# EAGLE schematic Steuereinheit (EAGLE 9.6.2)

## Sheet 1 of 5: PINS
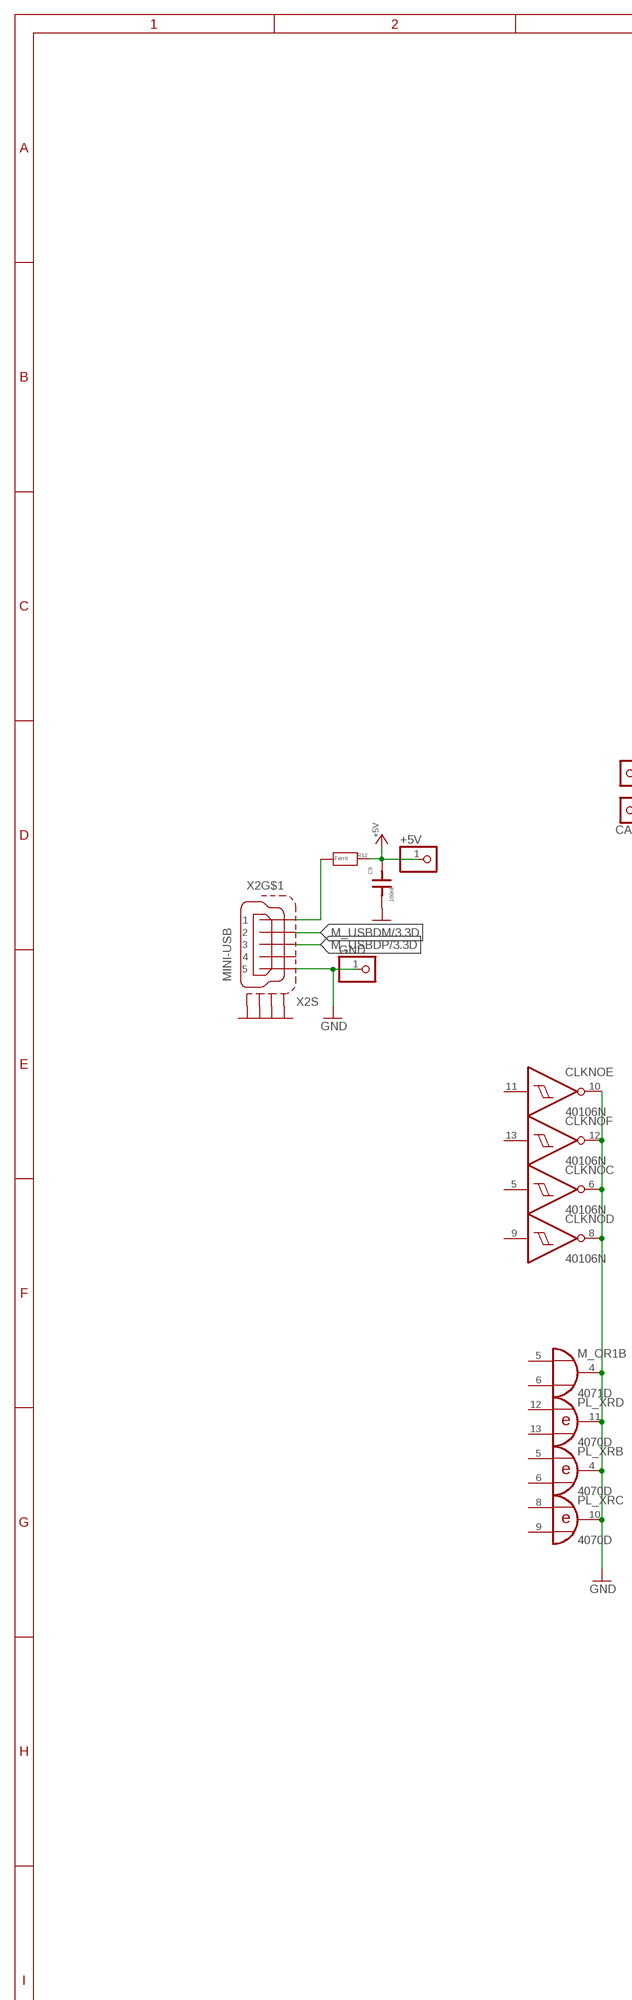
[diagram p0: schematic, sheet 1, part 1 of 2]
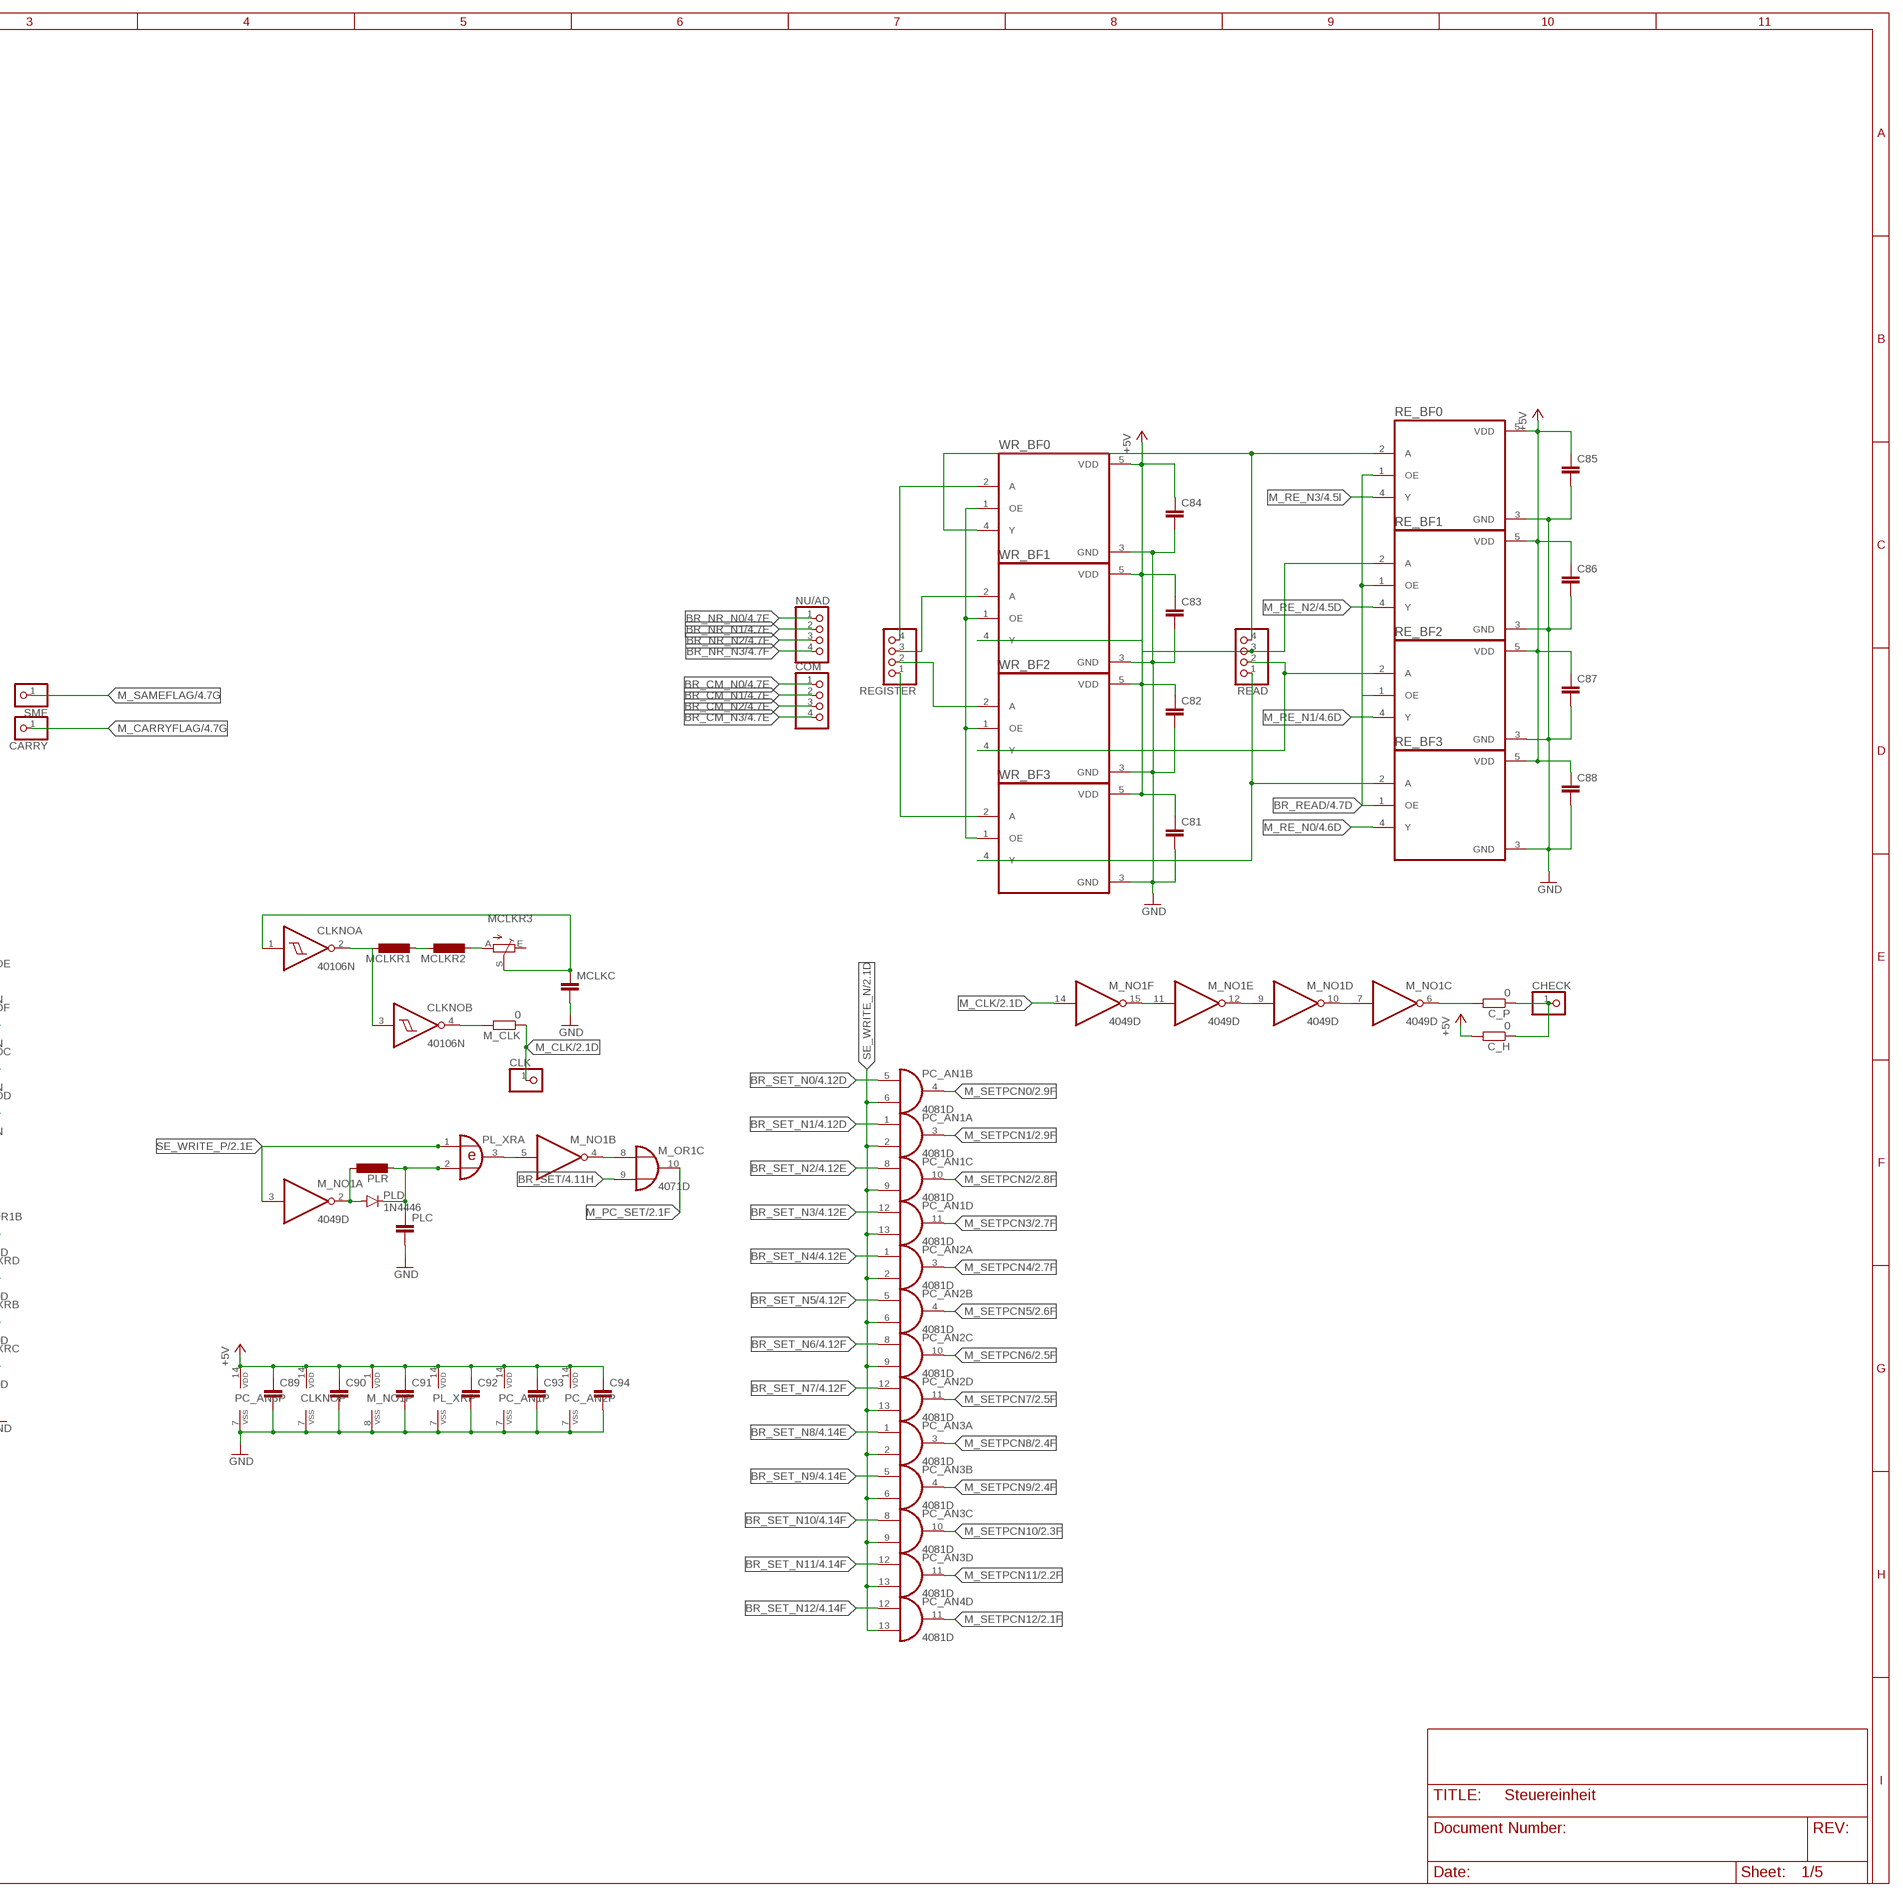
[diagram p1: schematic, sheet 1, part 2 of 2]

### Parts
+5V  PINHD-1X1  [1X01]
C9  100nF  C1  [0805F]
C81  C-EUC0805  [C0805]
C82  C-EUC0805  [C0805]
C83  C-EUC0805  [C0805]
C84  C-EUC0805  [C0805]
C85  C-EUC0805  [C0805]
C86  C-EUC0805  [C0805]
C87  C-EUC0805  [C0805]
C88  C-EUC0805  [C0805]
C89  C-EUC0805  [C0805]
C90  C-EUC0805  [C0805]
C91  C-EUC0805  [C0805]
C92  C-EUC0805  [C0805]
C93  C-EUC0805  [C0805]
C94  C-EUC0805  [C0805]
C_H  0  R-EU_R0805  [R0805]
C_P  0  R-EU_R0805  [R0805]
CARRY  PINHD-1X1  [1X01]
CHECK  PINHD-1X1  [1X01]
CLK  PINHD-1X1  [1X01]
CLKNO  40106N  [DIL14]
COM  PINHD-1X4  [1X04]
GND  PINHD-1X1  [1X01]
M_CLK  0  R-EU_R0805  [R0805]
M_NO1  4049D  [SO16]
M_OR1  4071D  [SO14]
MCLKC  C-EU025-030X050  [C025-030X050]
MCLKR1  L-EU0207/10  [0207/10]
MCLKR2  L-EU0207/10  [0207/10]
MCLKR3  TRIM_EU-CT6  [CT6]
NU/AD  PINHD-1X4  [1X04]
PC_AN1  4081D  [SO14]
PC_AN2  4081D  [SO14]
PC_AN3  4081D  [SO14]
PC_AN4  4081D  [SO14]
PL_XR  4070D  [SO14]
PLC  C-EU050-025X075  [C050-025X075]
PLD  1N4446  [DO35-10]
PLR  L-EU0207/10  [0207/10]
R12  Ferrit  R2  [1206]
RE_BF0  SN74LVC1G126DBVR  [SOT95P280X145-5N]
RE_BF1  SN74LVC1G126DBVR  [SOT95P280X145-5N]
RE_BF2  SN74LVC1G126DBVR  [SOT95P280X145-5N]
RE_BF3  SN74LVC1G126DBVR  [SOT95P280X145-5N]
READ  PINHD-1X4  [1X04]
REGISTER  PINHD-1X4  [1X04]
SMF  PINHD-1X1  [1X01]
WR_BF0  SN74LVC1G126DBVR  [SOT95P280X145-5N]
WR_BF1  SN74LVC1G126DBVR  [SOT95P280X145-5N]
WR_BF2  SN74LVC1G126DBVR  [SOT95P280X145-5N]
WR_BF3  SN74LVC1G126DBVR  [SOT95P280X145-5N]
X2  MINI-USB  MINI-USB-SCHIELD-32005-201  [32005-201]

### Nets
+5V: +5V.1 C9.2 C81.1 C82.1 C83.1 C84.1 C85.1 C86.1 C87.1 C88.1 C89.1 C90.1 C91.1 C92.1 C93.1 C94.1 C_H.2 CLKNO.14(P:VDD) M_NO1.1(P:VDD) PC_AN1.14(P:VDD) PC_AN2.14(P:VDD) PC_AN3.14(P:VDD) PL_XR.14(P:VDD) R12.2 RE_BF0.5(VDD) RE_BF1.5(VDD) RE_BF2.5(VDD) RE_BF3.5(VDD) WR_BF0.5(VDD) WR_BF1.5(VDD) WR_BF2.5(VDD) WR_BF3.5(VDD) ; also sheet 2,3,4,5
BR_CM_N0: COM.1 ; also sheet 4
BR_CM_N1: COM.2 ; also sheet 4
BR_CM_N2: COM.3 ; also sheet 4
BR_CM_N3: COM.4 ; also sheet 4
BR_NR_N0: NU/AD.1 ; also sheet 4
BR_NR_N1: NU/AD.2 ; also sheet 4
BR_NR_N2: NU/AD.3 ; also sheet 4
BR_NR_N3: NU/AD.4 ; also sheet 4
BR_READ: RE_BF0.1(OE) RE_BF1.1(OE) RE_BF2.1(OE) RE_BF3.1(OE) ; also sheet 4
BR_SET: M_OR1.9(C:I1) ; also sheet 4
BR_SET_N0: PC_AN1.5(B:I0) ; also sheet 4
BR_SET_N1: PC_AN1.1(A:I0) ; also sheet 4
BR_SET_N2: PC_AN1.8(C:I0) ; also sheet 4
BR_SET_N3: PC_AN1.12(D:I0) ; also sheet 4
BR_SET_N4: PC_AN2.1(A:I0) ; also sheet 4
BR_SET_N5: PC_AN2.5(B:I0) ; also sheet 4
BR_SET_N6: PC_AN2.8(C:I0) ; also sheet 4
BR_SET_N7: PC_AN2.12(D:I0) ; also sheet 4
BR_SET_N8: PC_AN3.1(A:I0) ; also sheet 4
BR_SET_N9: PC_AN3.5(B:I0) ; also sheet 4
BR_SET_N10: PC_AN3.8(C:I0) ; also sheet 4
BR_SET_N11: PC_AN3.12(D:I0) ; also sheet 4
BR_SET_N12: PC_AN4.12(D:I0) ; also sheet 4
GND: C9.1 C81.2 C82.2 C83.2 C84.2 C85.2 C86.2 C87.2 C88.2 C89.2 C90.2 C91.2 C92.2 C93.2 C94.2 CLKNO.6(C:O) CLKNO.7(P:VSS) CLKNO.8(D:O) CLKNO.10(E:O) CLKNO.12(F:O) GND.1 M_NO1.8(P:VSS) M_OR1.4(B:O) MCLKC.2 PC_AN1.7(P:VSS) PC_AN2.7(P:VSS) PC_AN3.7(P:VSS) PL_XR.4(B:O) PL_XR.7(P:VSS) PL_XR.10(C:O) PL_XR.11(D:O) PLC.2 RE_BF0.3(GND) RE_BF1.3(GND) RE_BF2.3(GND) RE_BF3.3(GND) WR_BF0.3(GND) WR_BF1.3(GND) WR_BF2.3(GND) WR_BF3.3(GND) X2.5 X2.M1(S:S1) X2.M2(S:S2) X2.M3(S:S3) X2.M4(S:S4) ; also sheet 2,3,4,5
M_CARRYFLAG: CARRY.1 ; also sheet 4
M_CLK: CLK.1 M_CLK.1 M_NO1.14(F:I) ; also sheet 2,3,4
M_PC_SET: M_OR1.10(C:O) ; also sheet 2
M_RE_N0: RE_BF3.4(Y) ; also sheet 4
M_RE_N1: RE_BF2.4(Y) ; also sheet 4
M_RE_N2: RE_BF1.4(Y) ; also sheet 4
M_RE_N3: RE_BF0.4(Y) ; also sheet 4
M_SAMEFLAG: SMF.1 ; also sheet 4
M_SETPCN0: PC_AN1.4(B:O) ; also sheet 2
M_SETPCN1: PC_AN1.3(A:O) ; also sheet 2
M_SETPCN2: PC_AN1.10(C:O) ; also sheet 2
M_SETPCN3: PC_AN1.11(D:O) ; also sheet 2
M_SETPCN4: PC_AN2.3(A:O) ; also sheet 2
M_SETPCN5: PC_AN2.4(B:O) ; also sheet 2
M_SETPCN6: PC_AN2.10(C:O) ; also sheet 2
M_SETPCN7: PC_AN2.11(D:O) ; also sheet 2
M_SETPCN8: PC_AN3.3(A:O) ; also sheet 2
M_SETPCN9: PC_AN3.4(B:O) ; also sheet 2
M_SETPCN10: PC_AN3.10(C:O) ; also sheet 2
M_SETPCN11: PC_AN3.11(D:O) ; also sheet 2
M_SETPCN12: PC_AN4.11(D:O) ; also sheet 2
M_USBDM: X2.2 ; also sheet 3
M_USBDP: X2.3 ; also sheet 3
N$177: CLKNO.4(B:O) M_CLK.2
N$179: C_P.2 M_NO1.6(C:O)
N$180: CLKNO.2(A:O) CLKNO.3(B:I) MCLKR1.1
N$181: C_H.1 C_P.1 CHECK.1
N$182: MCLKR2.2 MCLKR3.A
N$183: M_NO1.2(A:O) PLD.A PLR.1
N$184: PL_XR.2(A:I1) PLC.1 PLD.C PLR.2
N$186: RE_BF0.2(A) READ.4 WR_BF0.4(Y)
N$187: M_NO1.5(B:I) PL_XR.3(A:O)
N$188: RE_BF1.2(A) READ.3 WR_BF1.4(Y)
N$190: RE_BF2.2(A) READ.2 WR_BF2.4(Y)
N$192: RE_BF3.2(A) READ.1 WR_BF3.4(Y)
N$193: REGISTER.4 WR_BF0.2(A)
N$194: REGISTER.3 WR_BF1.2(A)
N$195: REGISTER.2 WR_BF2.2(A)
N$196: REGISTER.1 WR_BF3.2(A)
N$197: WR_BF0.1(OE) WR_BF1.1(OE) WR_BF2.1(OE) WR_BF3.1(OE)
N$198: M_NO1.4(B:O) M_OR1.8(C:I0)
N$199: CLKNO.1(A:I) MCLKC.1 MCLKR3.S
N$208: M_NO1.11(E:I) M_NO1.15(F:O)
N$209: M_NO1.9(D:I) M_NO1.12(E:O)
N$210: M_NO1.7(C:I) M_NO1.10(D:O)
N$212: MCLKR1.2 MCLKR2.1
SE_WRITE_N: PC_AN1.2(A:I1) PC_AN1.6(B:I1) PC_AN1.9(C:I1) PC_AN1.13(D:I1) PC_AN2.2(A:I1) PC_AN2.6(B:I1) PC_AN2.9(C:I1) PC_AN2.13(D:I1) PC_AN3.2(A:I1) PC_AN3.6(B:I1) PC_AN3.9(C:I1) PC_AN3.13(D:I1) PC_AN4.13(D:I1) ; also sheet 2,3,5
SE_WRITE_P: M_NO1.3(A:I) PL_XR.1(A:I0) ; also sheet 2,3,5
USB_4: R12.1 X2.1
Unconnected: CLKNO.5(C:I) CLKNO.9(D:I) CLKNO.11(E:I) CLKNO.13(F:I) M_OR1.5(B:I0) M_OR1.6(B:I1) MCLKR3.E PL_XR.5(B:I0) PL_XR.6(B:I1) PL_XR.8(C:I0) PL_XR.9(C:I1) PL_XR.12(D:I0) PL_XR.13(D:I1) X2.4

## Sheet 2 of 5: ProgrammCounter
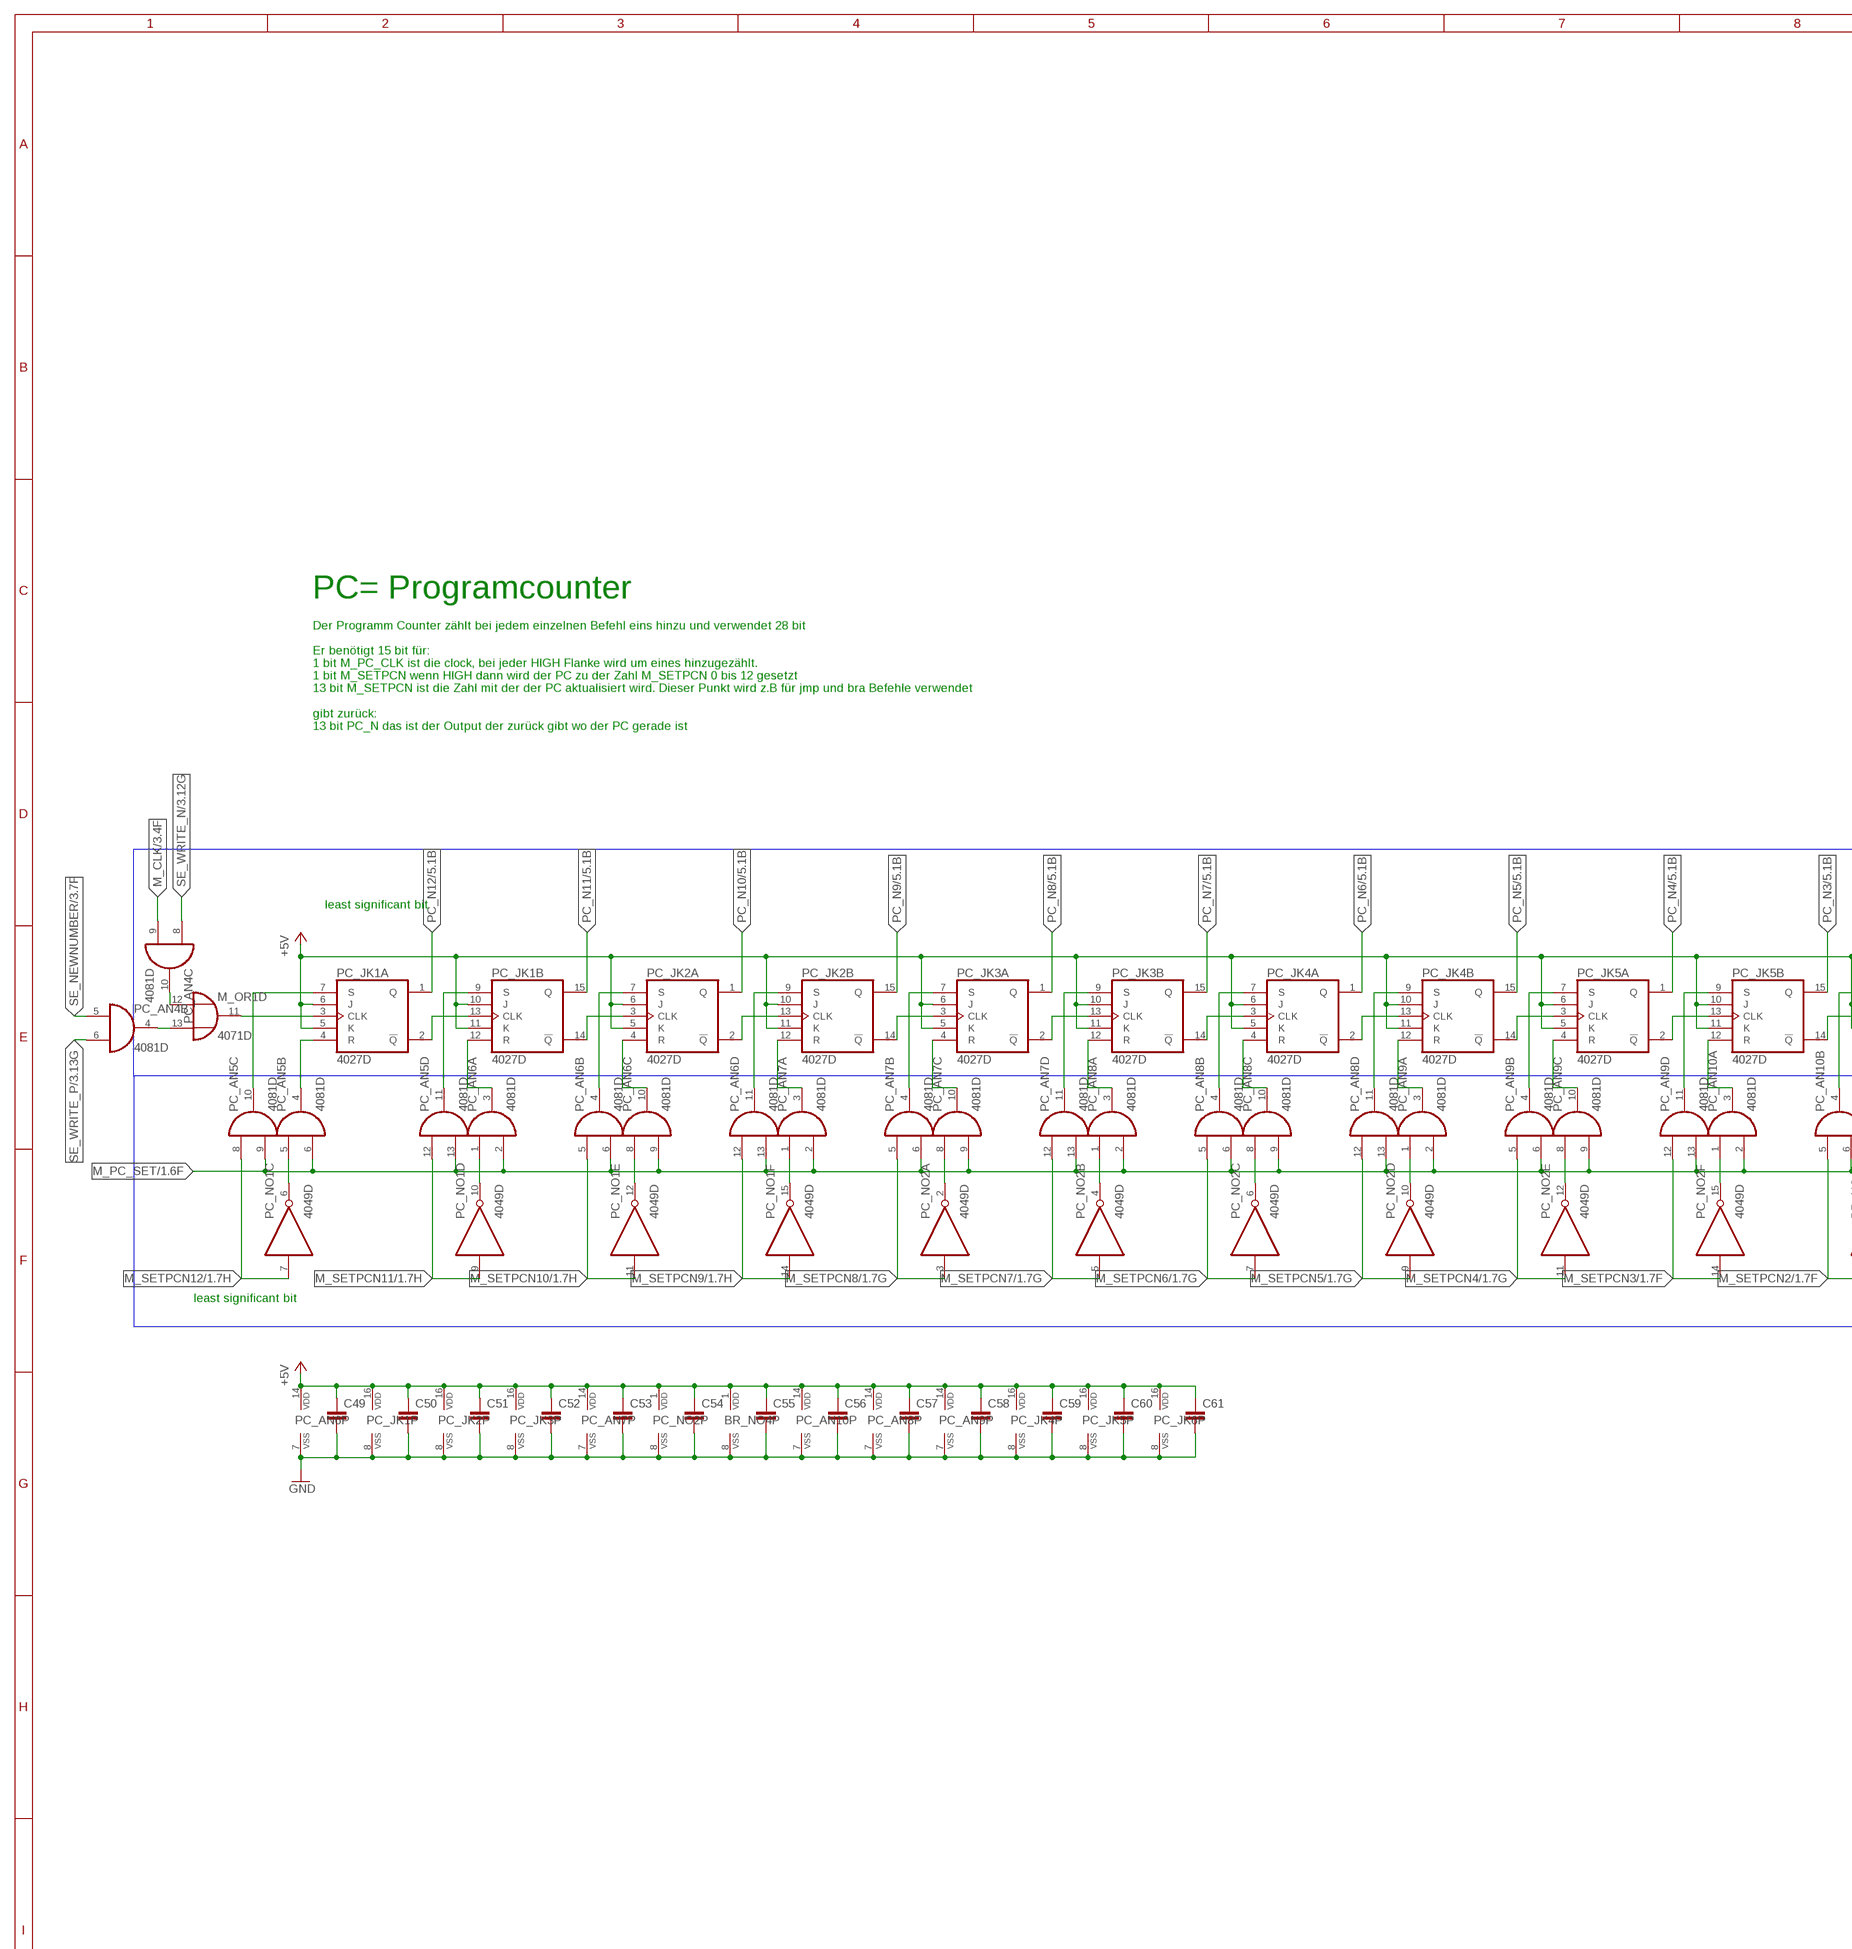
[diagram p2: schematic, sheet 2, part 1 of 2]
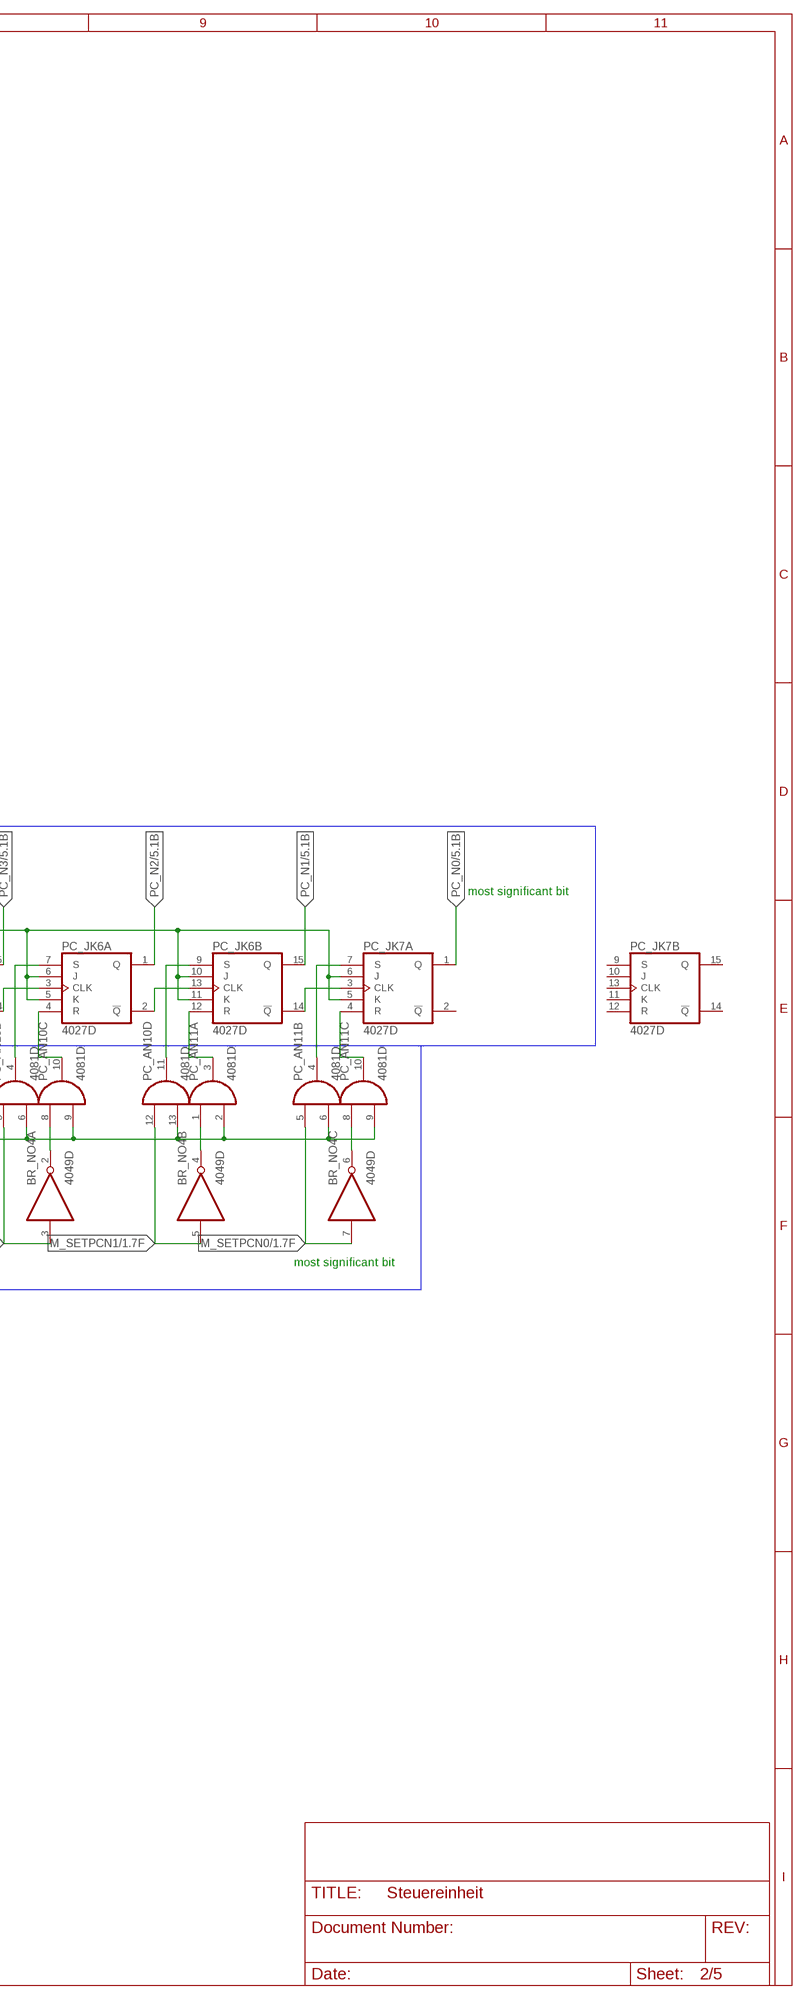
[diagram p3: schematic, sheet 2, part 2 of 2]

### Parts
BR_NO4  4049D  [SO16]
C49  C-EUC0805  [C0805]
C50  C-EUC0805  [C0805]
C51  C-EUC0805  [C0805]
C52  C-EUC0805  [C0805]
C53  C-EUC0805  [C0805]
C54  C-EUC0805  [C0805]
C55  C-EUC0805  [C0805]
C56  C-EUC0805  [C0805]
C57  C-EUC0805  [C0805]
C58  C-EUC0805  [C0805]
C59  C-EUC0805  [C0805]
C60  C-EUC0805  [C0805]
C61  C-EUC0805  [C0805]
PC_AN5  4081D  [SO14]
PC_AN6  4081D  [SO14]
PC_AN7  4081D  [SO14]
PC_AN8  4081D  [SO14]
PC_AN9  4081D  [SO14]
PC_AN10  4081D  [SO14]
PC_AN11  4081D  [SO14]
PC_JK1  4027D  [SO16]
PC_JK2  4027D  [SO16]
PC_JK3  4027D  [SO16]
PC_JK4  4027D  [SO16]
PC_JK5  4027D  [SO16]
PC_JK6  4027D  [SO16]
PC_JK7  4027D  [SO16]
PC_NO1  4049D  [SO16]
PC_NO2  4049D  [SO16]

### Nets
+5V: BR_NO4.1(P:VDD) C49.1 C50.1 C51.1 C52.1 C53.1 C54.1 C55.1 C56.1 C57.1 C58.1 C59.1 C60.1 C61.1 PC_AN6.14(P:VDD) PC_AN7.14(P:VDD) PC_AN8.14(P:VDD) PC_AN9.14(P:VDD) PC_AN10.14(P:VDD) PC_JK1.5(A:K) PC_JK1.6(A:J) PC_JK1.10(B:J) PC_JK1.11(B:K) PC_JK1.16(P:VDD) PC_JK2.5(A:K) PC_JK2.6(A:J) PC_JK2.10(B:J) PC_JK2.11(B:K) PC_JK2.16(P:VDD) PC_JK3.5(A:K) PC_JK3.6(A:J) PC_JK3.10(B:J) PC_JK3.11(B:K) PC_JK3.16(P:VDD) PC_JK4.5(A:K) PC_JK4.6(A:J) PC_JK4.10(B:J) PC_JK4.11(B:K) PC_JK4.16(P:VDD) PC_JK5.5(A:K) PC_JK5.6(A:J) PC_JK5.10(B:J) PC_JK5.11(B:K) PC_JK5.16(P:VDD) PC_JK6.5(A:K) PC_JK6.6(A:J) PC_JK6.10(B:J) PC_JK6.11(B:K) PC_JK6.16(P:VDD) PC_JK7.5(A:K) PC_JK7.6(A:J) PC_NO2.1(P:VDD) ; also sheet 1,3,4,5
GND: BR_NO4.8(P:VSS) C49.2 C50.2 C51.2 C52.2 C53.2 C54.2 C55.2 C56.2 C57.2 C58.2 C59.2 C60.2 C61.2 PC_AN6.7(P:VSS) PC_AN7.7(P:VSS) PC_AN8.7(P:VSS) PC_AN9.7(P:VSS) PC_AN10.7(P:VSS) PC_JK1.8(P:VSS) PC_JK2.8(P:VSS) PC_JK3.8(P:VSS) PC_JK4.8(P:VSS) PC_JK5.8(P:VSS) PC_JK6.8(P:VSS) PC_NO2.8(P:VSS) ; also sheet 1,3,4,5
M_CLK: PC_AN4.9(C:I1) ; also sheet 1,3,4
M_PC_SET: PC_AN5.6(B:I1) PC_AN5.9(C:I1) PC_AN5.13(D:I1) PC_AN6.2(A:I1) PC_AN6.6(B:I1) PC_AN6.9(C:I1) PC_AN6.13(D:I1) PC_AN7.2(A:I1) PC_AN7.6(B:I1) PC_AN7.9(C:I1) PC_AN7.13(D:I1) PC_AN8.2(A:I1) PC_AN8.6(B:I1) PC_AN8.9(C:I1) PC_AN8.13(D:I1) PC_AN9.2(A:I1) PC_AN9.6(B:I1) PC_AN9.9(C:I1) PC_AN9.13(D:I1) PC_AN10.2(A:I1) PC_AN10.6(B:I1) PC_AN10.9(C:I1) PC_AN10.13(D:I1) PC_AN11.2(A:I1) PC_AN11.6(B:I1) PC_AN11.9(C:I1) ; also sheet 1
M_SETPCN0: BR_NO4.7(C:I) PC_AN11.5(B:I0) ; also sheet 1
M_SETPCN1: BR_NO4.5(B:I) PC_AN10.12(D:I0) ; also sheet 1
M_SETPCN2: BR_NO4.3(A:I) PC_AN10.5(B:I0) ; also sheet 1
M_SETPCN3: PC_AN9.12(D:I0) PC_NO2.14(F:I) ; also sheet 1
M_SETPCN4: PC_AN9.5(B:I0) PC_NO2.11(E:I) ; also sheet 1
M_SETPCN5: PC_AN8.12(D:I0) PC_NO2.9(D:I) ; also sheet 1
M_SETPCN6: PC_AN8.5(B:I0) PC_NO2.7(C:I) ; also sheet 1
M_SETPCN7: PC_AN7.12(D:I0) PC_NO2.5(B:I) ; also sheet 1
M_SETPCN8: PC_AN7.5(B:I0) PC_NO2.3(A:I) ; also sheet 1
M_SETPCN9: PC_AN6.12(D:I0) PC_NO1.14(F:I) ; also sheet 1
M_SETPCN10: PC_AN6.5(B:I0) PC_NO1.11(E:I) ; also sheet 1
M_SETPCN11: PC_AN5.12(D:I0) PC_NO1.9(D:I) ; also sheet 1
M_SETPCN12: PC_AN5.8(C:I0) PC_NO1.7(C:I) ; also sheet 1
N$40: PC_JK1.2(A:!Q) PC_JK1.13(B:CLK)
N$50: PC_JK1.14(B:!Q) PC_JK2.3(A:CLK)
N$51: PC_JK2.2(A:!Q) PC_JK2.13(B:CLK)
N$52: PC_JK2.14(B:!Q) PC_JK3.3(A:CLK)
N$53: PC_JK3.2(A:!Q) PC_JK3.13(B:CLK)
N$54: PC_JK3.14(B:!Q) PC_JK4.3(A:CLK)
N$55: PC_JK4.2(A:!Q) PC_JK4.13(B:CLK)
N$56: PC_JK4.14(B:!Q) PC_JK5.3(A:CLK)
N$57: PC_JK5.2(A:!Q) PC_JK5.13(B:CLK)
N$58: PC_JK5.14(B:!Q) PC_JK6.3(A:CLK)
N$59: PC_JK6.2(A:!Q) PC_JK6.13(B:CLK)
N$60: PC_JK6.14(B:!Q) PC_JK7.3(A:CLK)
N$62: PC_AN5.10(C:O) PC_JK1.7(A:S)
N$63: PC_AN5.4(B:O) PC_JK1.4(A:R)
N$64: PC_AN5.11(D:O) PC_JK1.9(B:S)
N$65: PC_AN6.3(A:O) PC_JK1.12(B:R)
N$66: PC_AN6.4(B:O) PC_JK2.7(A:S)
N$67: PC_AN6.10(C:O) PC_JK2.4(A:R)
N$68: PC_AN6.11(D:O) PC_JK2.9(B:S)
N$69: PC_AN7.3(A:O) PC_JK2.12(B:R)
N$70: PC_AN7.4(B:O) PC_JK3.7(A:S)
N$71: PC_AN7.10(C:O) PC_JK3.4(A:R)
N$72: PC_AN7.11(D:O) PC_JK3.9(B:S)
N$73: PC_AN8.3(A:O) PC_JK3.12(B:R)
N$74: PC_AN8.4(B:O) PC_JK4.7(A:S)
N$75: PC_AN8.10(C:O) PC_JK4.4(A:R)
N$76: PC_AN8.11(D:O) PC_JK4.9(B:S)
N$77: PC_AN9.3(A:O) PC_JK4.12(B:R)
N$78: PC_AN9.4(B:O) PC_JK5.7(A:S)
N$79: PC_AN9.10(C:O) PC_JK5.4(A:R)
N$80: PC_AN9.11(D:O) PC_JK5.9(B:S)
N$81: PC_AN10.3(A:O) PC_JK5.12(B:R)
N$82: PC_AN10.4(B:O) PC_JK6.7(A:S)
N$83: PC_AN10.10(C:O) PC_JK6.4(A:R)
N$84: PC_AN10.11(D:O) PC_JK6.9(B:S)
N$85: PC_AN11.3(A:O) PC_JK6.12(B:R)
N$86: PC_AN11.4(B:O) PC_JK7.7(A:S)
N$87: PC_AN11.10(C:O) PC_JK7.4(A:R)
N$88: PC_AN5.5(B:I0) PC_NO1.6(C:O)
N$91: PC_AN6.1(A:I0) PC_NO1.10(D:O)
N$93: PC_AN6.8(C:I0) PC_NO1.12(E:O)
N$95: PC_AN7.1(A:I0) PC_NO1.15(F:O)
N$97: PC_AN7.8(C:I0) PC_NO2.2(A:O)
N$99: PC_AN8.1(A:I0) PC_NO2.4(B:O)
N$101: PC_AN8.8(C:I0) PC_NO2.6(C:O)
N$103: PC_AN9.1(A:I0) PC_NO2.10(D:O)
N$105: PC_AN9.8(C:I0) PC_NO2.12(E:O)
N$107: PC_AN10.1(A:I0) PC_NO2.15(F:O)
N$109: BR_NO4.2(A:O) PC_AN10.8(C:I0)
N$111: BR_NO4.4(B:O) PC_AN11.1(A:I0)
N$113: BR_NO4.6(C:O) PC_AN11.8(C:I0)
N$185: M_OR1.13(D:I1) PC_AN4.4(B:O)
N$189: M_OR1.11(D:O) PC_JK1.3(A:CLK)
N$191: M_OR1.12(D:I0) PC_AN4.10(C:O)
PC_N0: PC_JK7.1(A:Q) ; also sheet 5
PC_N1: PC_JK6.15(B:Q) ; also sheet 5
PC_N2: PC_JK6.1(A:Q) ; also sheet 5
PC_N3: PC_JK5.15(B:Q) ; also sheet 5
PC_N4: PC_JK5.1(A:Q) ; also sheet 5
PC_N5: PC_JK4.15(B:Q) ; also sheet 5
PC_N6: PC_JK4.1(A:Q) ; also sheet 5
PC_N7: PC_JK3.15(B:Q) ; also sheet 5
PC_N8: PC_JK3.1(A:Q) ; also sheet 5
PC_N9: PC_JK2.15(B:Q) ; also sheet 5
PC_N10: PC_JK2.1(A:Q) ; also sheet 5
PC_N11: PC_JK1.15(B:Q) ; also sheet 5
PC_N12: PC_JK1.1(A:Q) ; also sheet 5
SE_NEWNUMBER: PC_AN4.5(B:I0) ; also sheet 3
SE_WRITE_N: PC_AN4.8(C:I0) ; also sheet 1,3,5
SE_WRITE_P: PC_AN4.6(B:I1) ; also sheet 1,3,5
Unconnected: PC_JK7.2(A:!Q) PC_JK7.9(B:S) PC_JK7.10(B:J) PC_JK7.11(B:K) PC_JK7.12(B:R) PC_JK7.13(B:CLK) PC_JK7.14(B:!Q) PC_JK7.15(B:Q)

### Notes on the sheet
- PC= Programcounter
- Der Programm Counter zählt bei jedem einzelnen Befehl eins hinzu und verwendet 28 bit
  
  Er benötigt 15 bit für:
  1 bit M_PC_CLK ist die clock, bei jeder HIGH Flanke wird um eines hinzugezählt.
  1 bit M_SETPCN wenn HIGH dann wird der PC zu der Zahl M_SETPCN 0 bis 12 gesetzt
  13 bit M_SETPCN ist die Zahl mit der der PC aktualisiert wird. Dieser Punkt wird z.B für jmp und bra Befehle verwendet
  
  gibt zurück:
  13 bit PC_N das ist der Output der zurück gibt wo der PC gerade ist
- least significant bit
- most significant bit
- least significant bit | most significant bit

## Sheet 3 of 5: Serielle
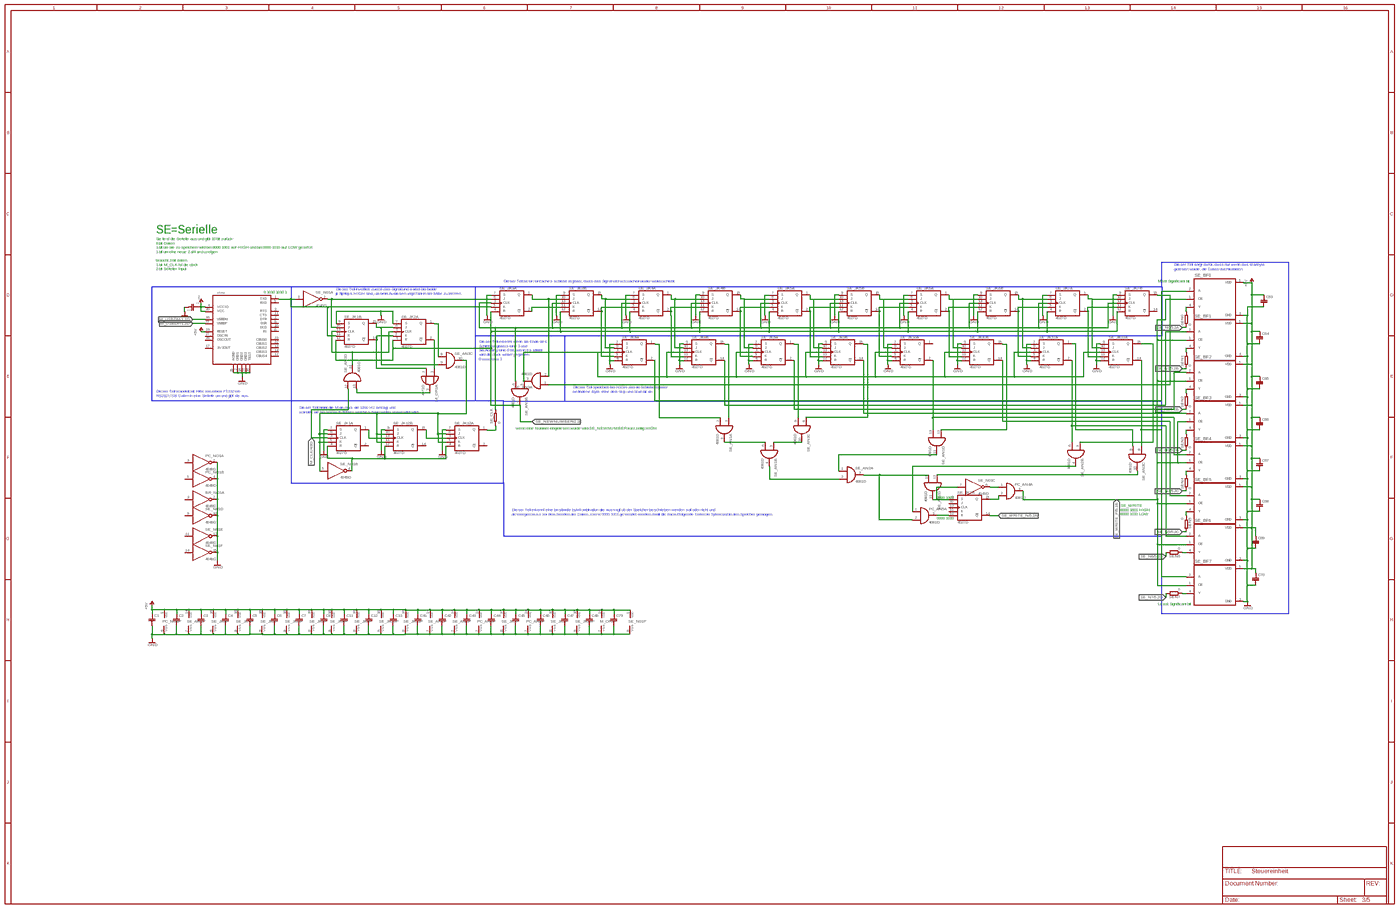
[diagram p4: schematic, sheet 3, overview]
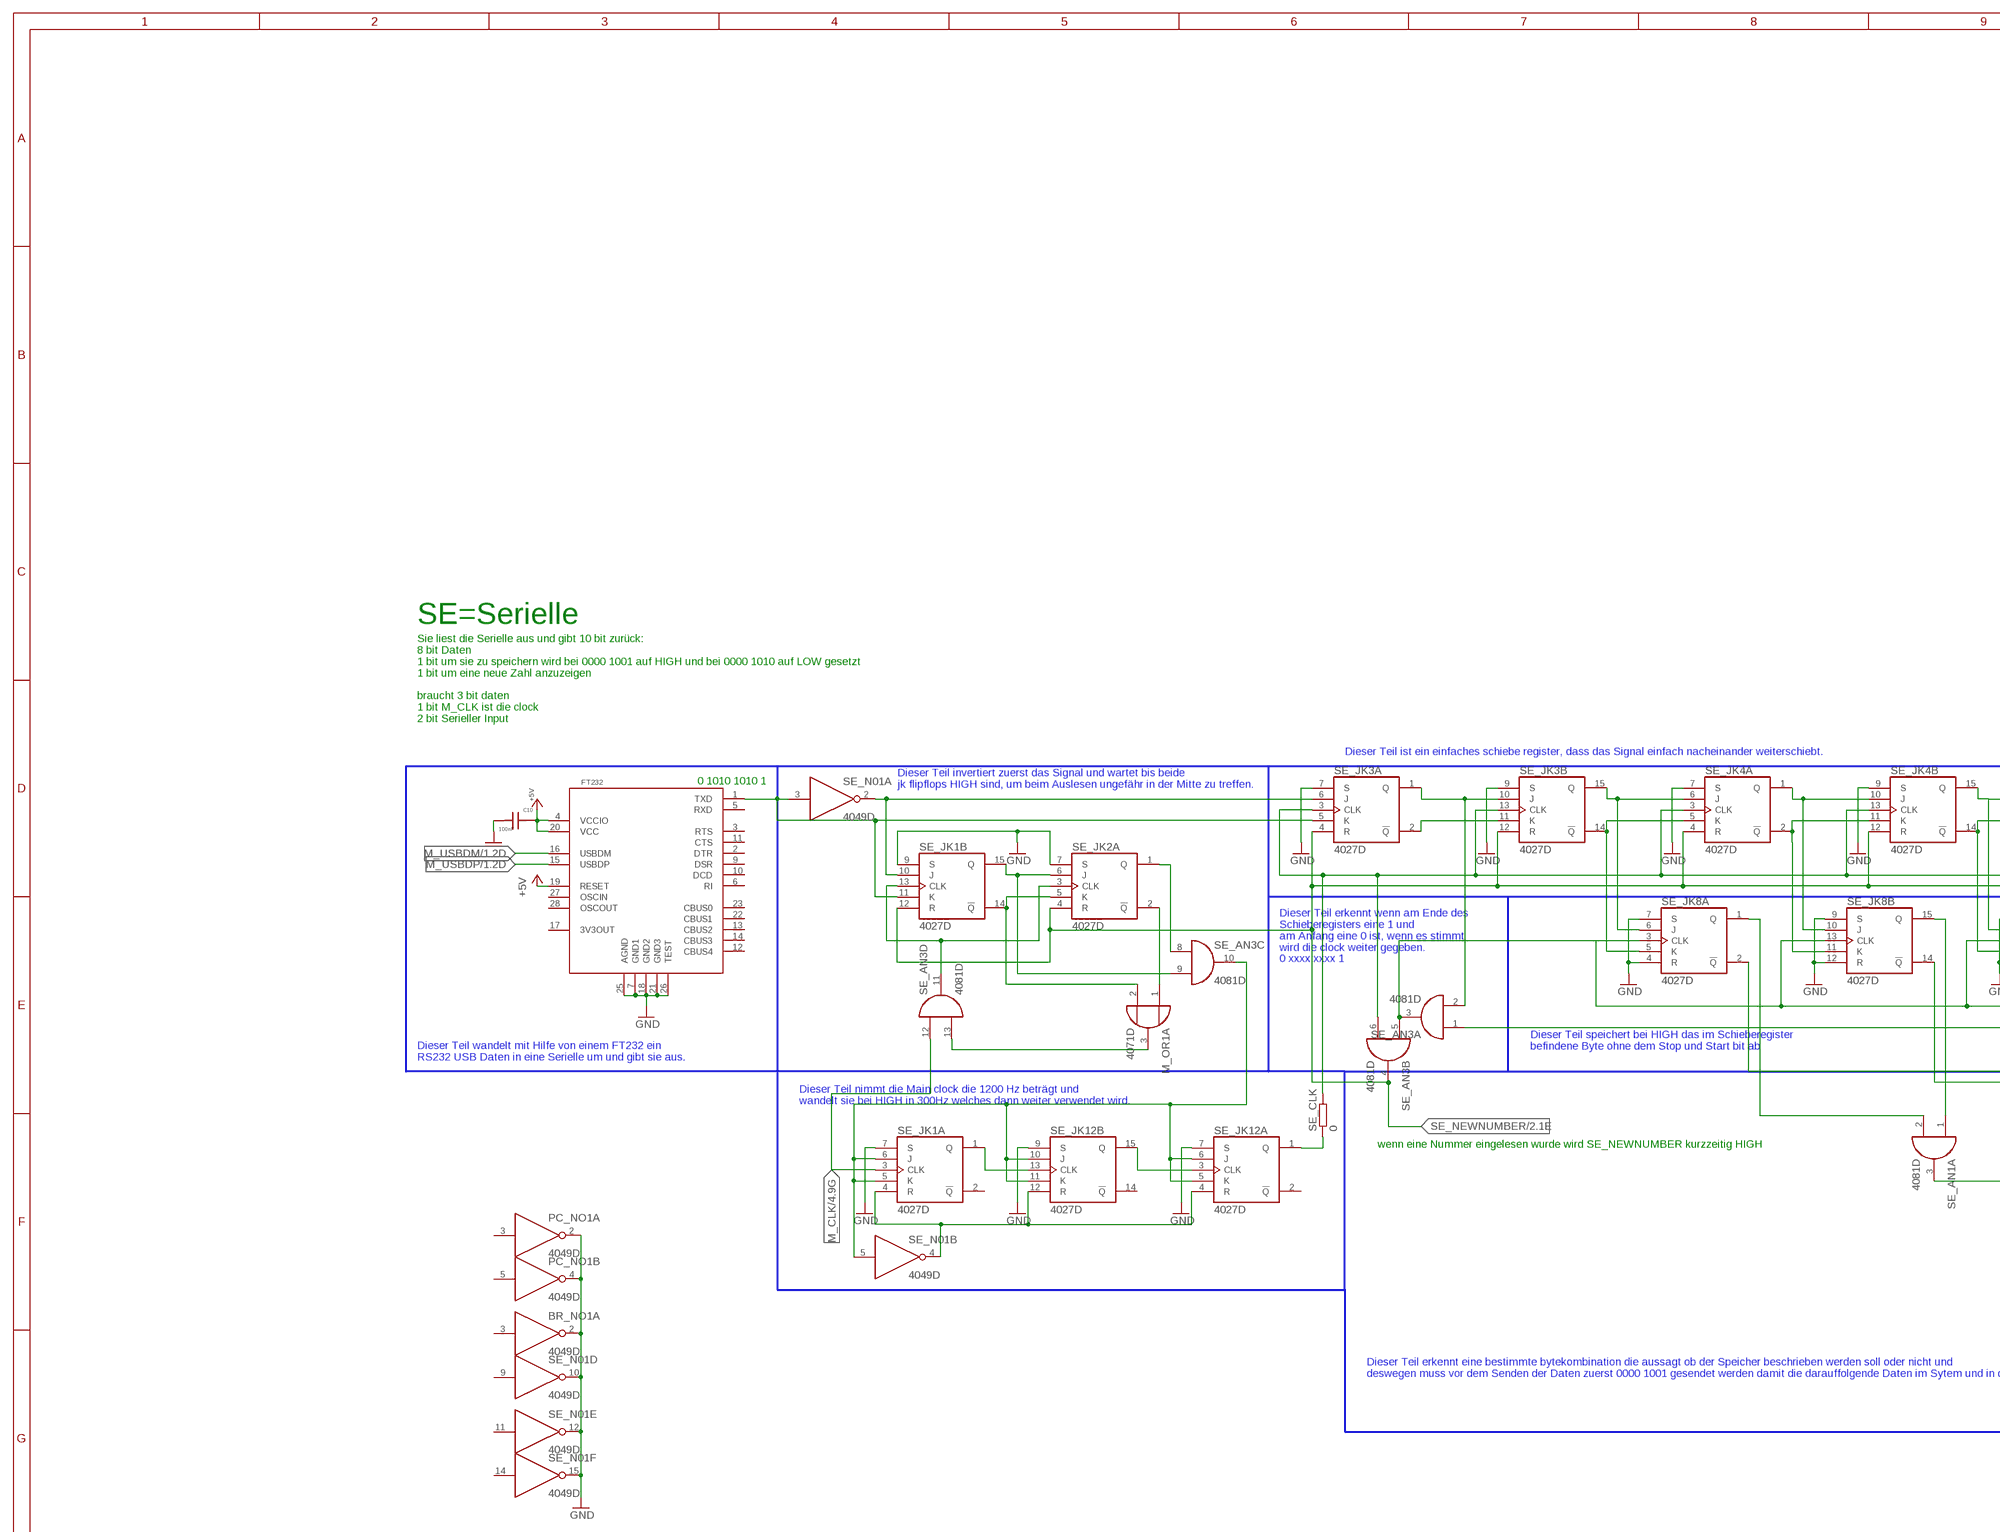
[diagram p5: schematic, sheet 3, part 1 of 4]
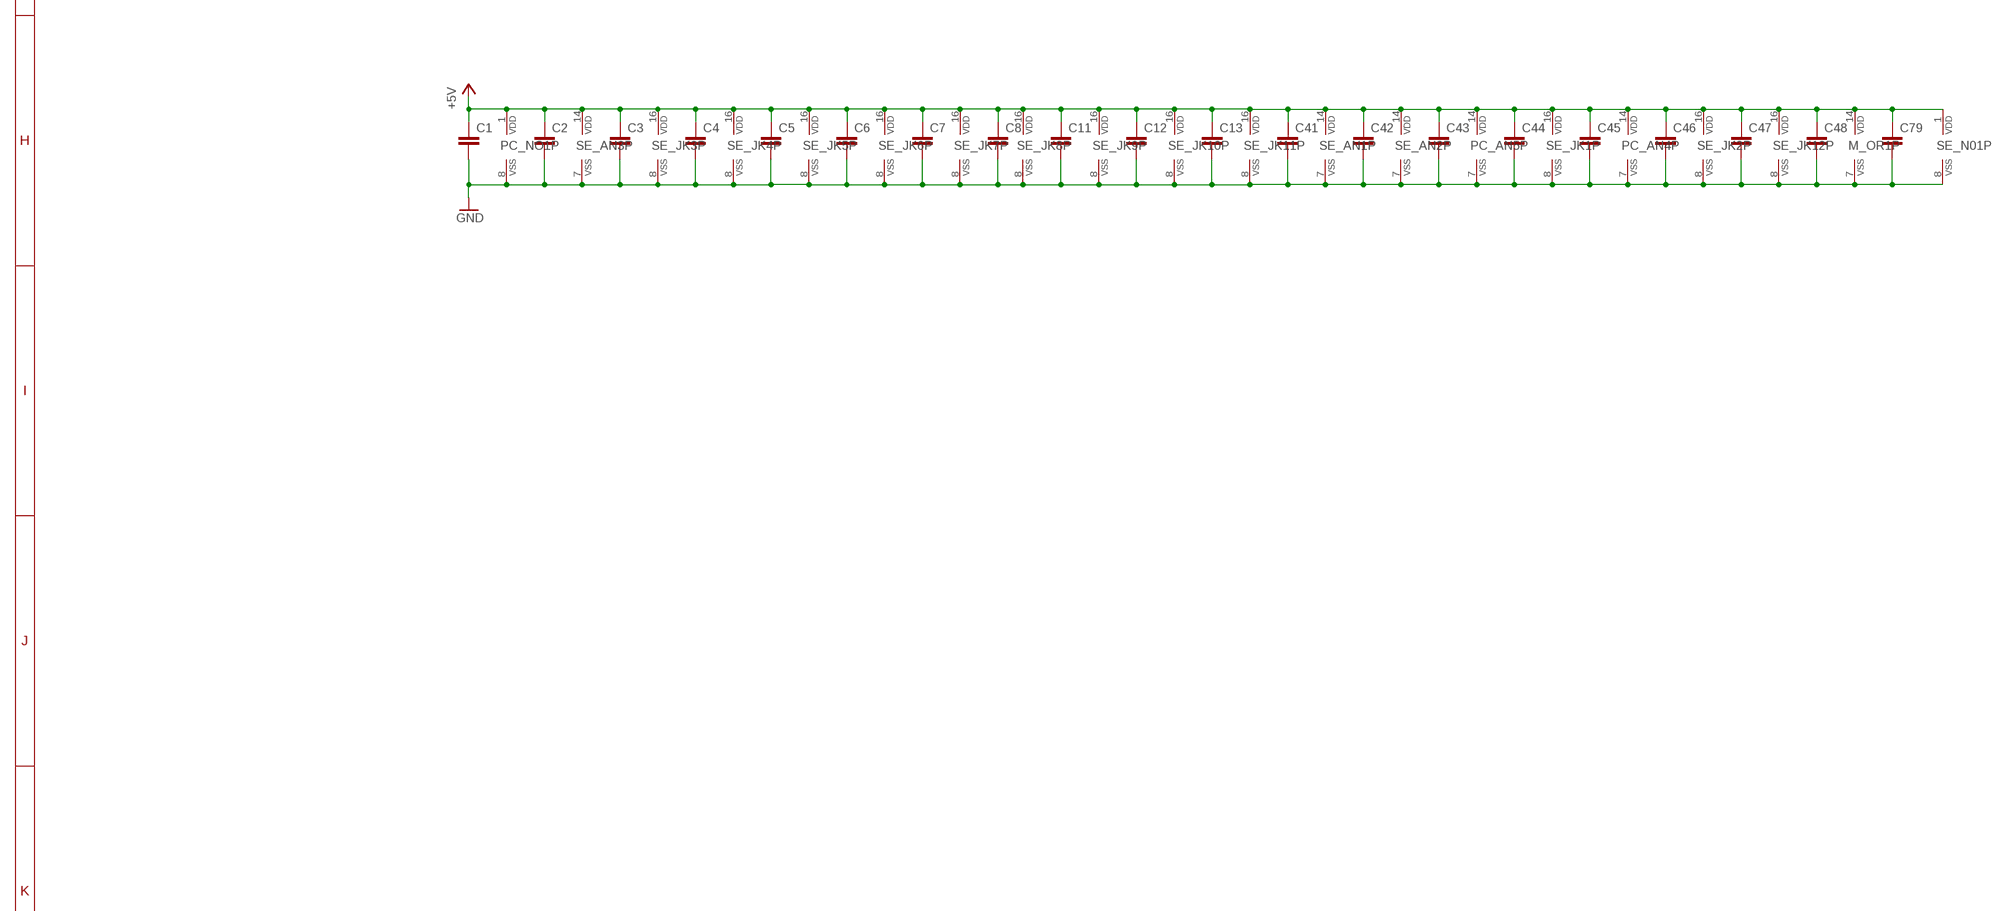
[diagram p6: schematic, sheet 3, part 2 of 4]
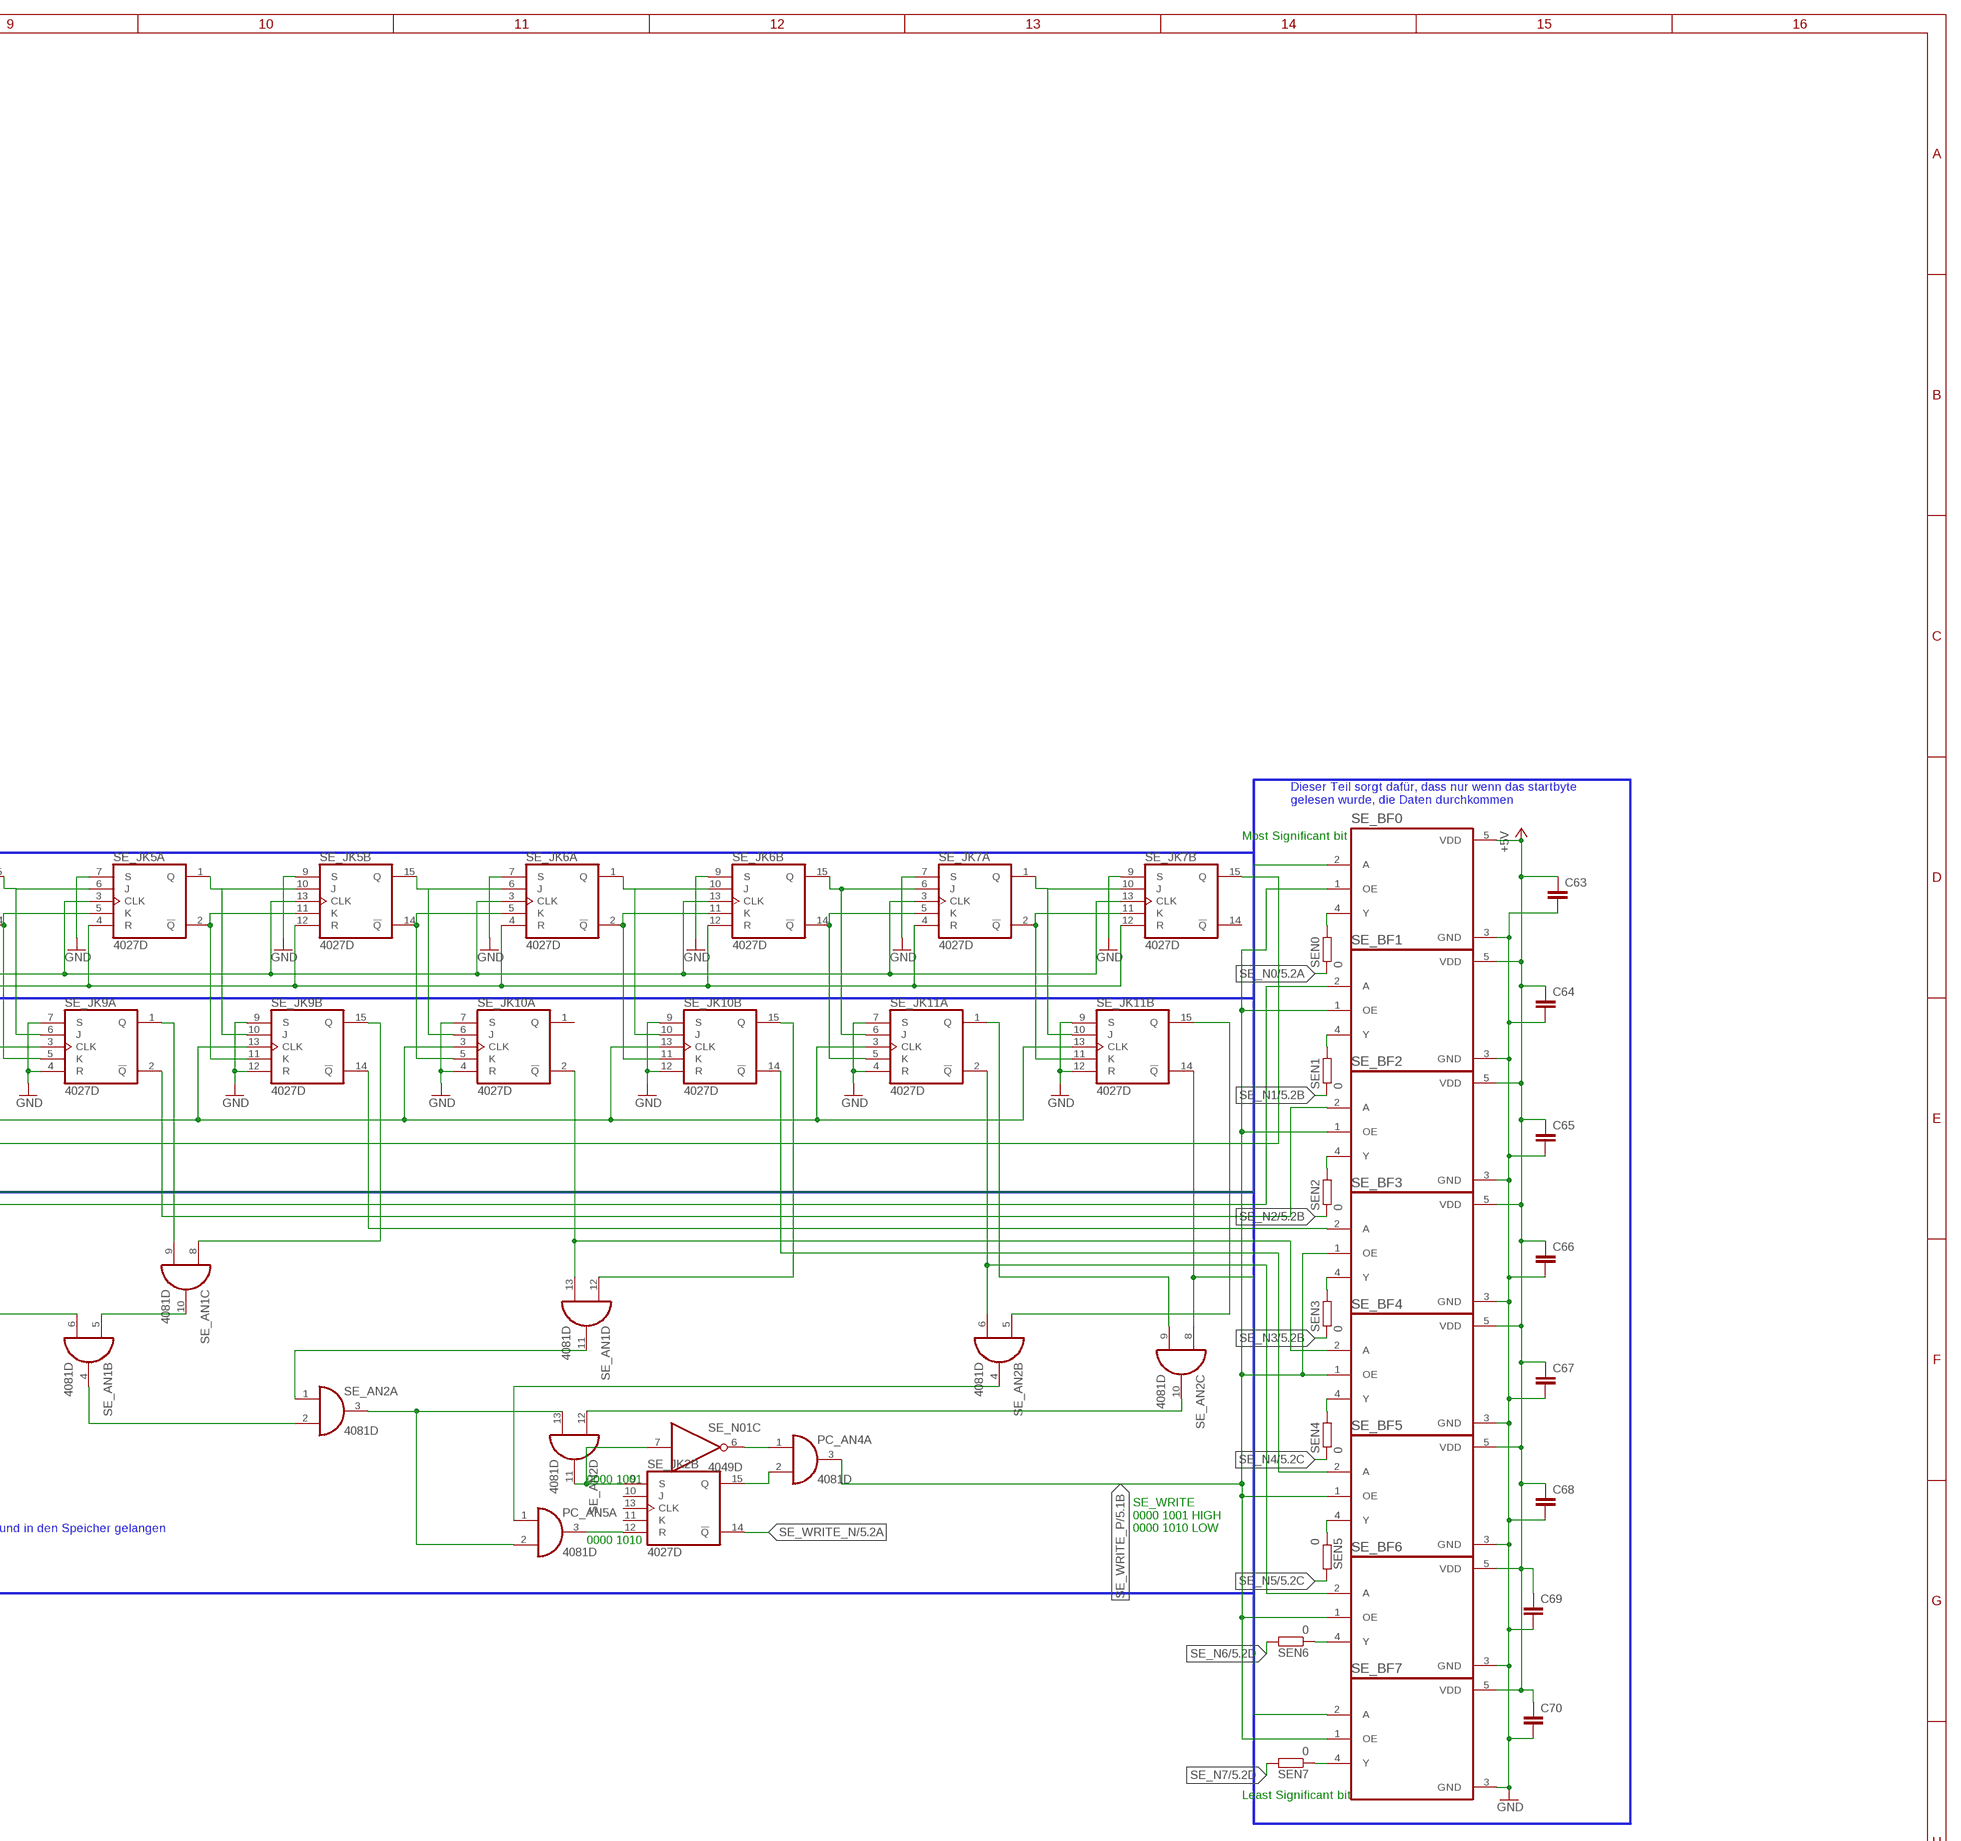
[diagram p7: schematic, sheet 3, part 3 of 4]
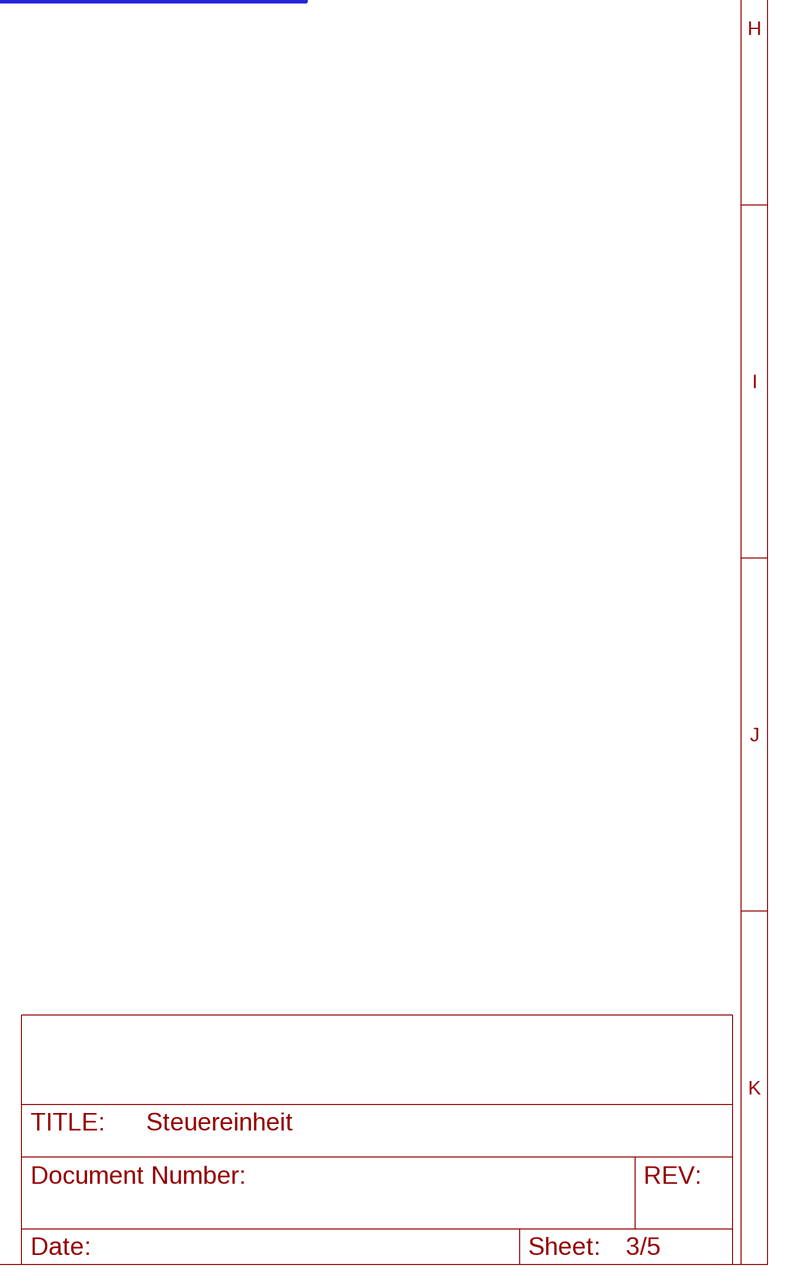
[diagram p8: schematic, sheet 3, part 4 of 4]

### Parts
BR_NO1  4049D  [SO16]
C1  C-EUC0805  [C0805]
C2  C-EUC0805  [C0805]
C3  C-EUC0805  [C0805]
C4  C-EUC0805  [C0805]
C5  C-EUC0805  [C0805]
C6  C-EUC0805  [C0805]
C7  C-EUC0805  [C0805]
C8  C-EUC0805  [C0805]
C10  100nF  C1  [0805F]
C11  C-EUC0805  [C0805]
C12  C-EUC0805  [C0805]
C13  C-EUC0805  [C0805]
C41  C-EUC0805  [C0805]
C42  C-EUC0805  [C0805]
C43  C-EUC0805  [C0805]
C44  C-EUC0805  [C0805]
C45  C-EUC0805  [C0805]
C46  C-EUC0805  [C0805]
C47  C-EUC0805  [C0805]
C48  C-EUC0805  [C0805]
C63  C-EUC0805  [C0805]
C64  C-EUC0805  [C0805]
C65  C-EUC0805  [C0805]
C66  C-EUC0805  [C0805]
C67  C-EUC0805  [C0805]
C68  C-EUC0805  [C0805]
C69  C-EUC0805  [C0805]
C70  C-EUC0805  [C0805]
C79  C-EUC0805  [C0805]
FT232  FTDI232RL  [SSOP28]
SE_AN1  4081D  [SO14]
SE_AN2  4081D  [SO14]
SE_AN3  4081D  [SO14]
SE_BF0  SN74LVC1G126DBVR  [SOT95P280X145-5N]
SE_BF1  SN74LVC1G126DBVR  [SOT95P280X145-5N]
SE_BF2  SN74LVC1G126DBVR  [SOT95P280X145-5N]
SE_BF3  SN74LVC1G126DBVR  [SOT95P280X145-5N]
SE_BF4  SN74LVC1G126DBVR  [SOT95P280X145-5N]
SE_BF5  SN74LVC1G126DBVR  [SOT95P280X145-5N]
SE_BF6  SN74LVC1G126DBVR  [SOT95P280X145-5N]
SE_BF7  SN74LVC1G126DBVR  [SOT95P280X145-5N]
SE_CLK  0  R-EU_R0805  [R0805]
SE_JK1  4027D  [SO16]
SE_JK2  4027D  [SO16]
SE_JK3  4027D  [SO16]
SE_JK4  4027D  [SO16]
SE_JK5  4027D  [SO16]
SE_JK6  4027D  [SO16]
SE_JK7  4027D  [SO16]
SE_JK8  4027D  [SO16]
SE_JK9  4027D  [SO16]
SE_JK10  4027D  [SO16]
SE_JK11  4027D  [SO16]
SE_JK12  4027D  [SO16]
SE_N01  4049D  [SO16]
SEN0  0  R-EU_R0805  [R0805]
SEN1  0  R-EU_R0805  [R0805]
SEN2  0  R-EU_R0805  [R0805]
SEN3  0  R-EU_R0805  [R0805]
SEN4  0  R-EU_R0805  [R0805]
SEN5  0  R-EU_R0805  [R0805]
SEN6  0  R-EU_R0805  [R0805]
SEN7  0  R-EU_R0805  [R0805]

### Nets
+5V: C1.1 C2.1 C3.1 C4.1 C5.1 C6.1 C7.1 C8.1 C10.2 C11.1 C12.1 C13.1 C41.1 C42.1 C43.1 C44.1 C45.1 C46.1 C47.1 C48.1 C63.1 C64.1 C65.1 C66.1 C67.1 C68.1 C69.1 C70.1 C79.1 FT232.4(VCCIO) FT232.19(RESET) FT232.20(VCC) M_OR1.14(P:VDD) PC_AN4.14(P:VDD) PC_AN5.14(P:VDD) PC_NO1.1(P:VDD) SE_AN1.14(P:VDD) SE_AN2.14(P:VDD) SE_AN3.14(P:VDD) SE_BF0.5(VDD) SE_BF1.5(VDD) SE_BF2.5(VDD) SE_BF3.5(VDD) SE_BF4.5(VDD) SE_BF5.5(VDD) SE_BF6.5(VDD) SE_BF7.5(VDD) SE_JK1.16(P:VDD) SE_JK2.16(P:VDD) SE_JK3.16(P:VDD) SE_JK4.16(P:VDD) SE_JK5.16(P:VDD) SE_JK6.16(P:VDD) SE_JK7.16(P:VDD) SE_JK8.16(P:VDD) SE_JK9.16(P:VDD) SE_JK10.16(P:VDD) SE_JK11.16(P:VDD) SE_JK12.16(P:VDD) SE_N01.1(P:VDD) ; also sheet 1,2,4,5
GND: BR_NO1.2(A:O) C1.2 C2.2 C3.2 C4.2 C5.2 C6.2 C7.2 C8.2 C10.1 C11.2 C12.2 C13.2 C41.2 C42.2 C43.2 C44.2 C45.2 C46.2 C47.2 C48.2 C63.2 C64.2 C65.2 C66.2 C67.2 C68.2 C69.2 C70.2 C79.2 FT232.7(GND1) FT232.18(GND2) FT232.21(GND3) FT232.25(AGND) FT232.26(TEST) M_OR1.7(P:VSS) PC_AN4.7(P:VSS) PC_AN5.7(P:VSS) PC_NO1.2(A:O) PC_NO1.4(B:O) PC_NO1.8(P:VSS) SE_AN1.7(P:VSS) SE_AN2.7(P:VSS) SE_AN3.7(P:VSS) SE_BF0.3(GND) SE_BF1.3(GND) SE_BF2.3(GND) SE_BF3.3(GND) SE_BF4.3(GND) SE_BF5.3(GND) SE_BF6.3(GND) SE_BF7.3(GND) SE_JK1.7(A:S) SE_JK1.8(P:VSS) SE_JK1.9(B:S) SE_JK2.7(A:S) SE_JK2.8(P:VSS) SE_JK3.7(A:S) SE_JK3.8(P:VSS) SE_JK3.9(B:S) SE_JK4.7(A:S) SE_JK4.8(P:VSS) SE_JK4.9(B:S) SE_JK5.7(A:S) SE_JK5.8(P:VSS) SE_JK5.9(B:S) SE_JK6.7(A:S) SE_JK6.8(P:VSS) SE_JK6.9(B:S) SE_JK7.7(A:S) SE_JK7.8(P:VSS) SE_JK7.9(B:S) SE_JK8.4(A:R) SE_JK8.7(A:S) SE_JK8.8(P:VSS) SE_JK8.9(B:S) SE_JK8.12(B:R) SE_JK9.4(A:R) SE_JK9.7(A:S) SE_JK9.8(P:VSS) SE_JK9.9(B:S) SE_JK9.12(B:R) SE_JK10.4(A:R) SE_JK10.7(A:S) SE_JK10.8(P:VSS) SE_JK10.9(B:S) SE_JK10.12(B:R) SE_JK11.4(A:R) SE_JK11.7(A:S) SE_JK11.8(P:VSS) SE_JK11.9(B:S) SE_JK11.12(B:R) SE_JK12.7(A:S) SE_JK12.8(P:VSS) SE_JK12.9(B:S) SE_N01.8(P:VSS) SE_N01.10(D:O) SE_N01.12(E:O) SE_N01.15(F:O) ; also sheet 1,2,4,5
M_CLK: SE_AN3.12(D:I0) SE_JK1.3(A:CLK) ; also sheet 1,2,4
M_USBDM: FT232.16(USBDM) ; also sheet 1
M_USBDP: FT232.15(USBDP) ; also sheet 1
N$1: SE_AN3.9(C:I1) SE_JK1.15(B:Q) SE_JK2.6(A:J)
N$2: FT232.1(TXD) SE_JK1.11(B:K) SE_JK3.5(A:K) SE_N01.3(A:I)
N$3: SE_JK1.10(B:J) SE_JK3.6(A:J) SE_N01.2(A:O)
N$4: SE_JK1.1(A:Q) SE_JK12.13(B:CLK)
N$5: SE_AN3.2(A:I1) SE_JK3.1(A:Q) SE_JK3.10(B:J)
N$6: SE_JK3.2(A:!Q) SE_JK3.11(B:K)
N$7: M_OR1.3(A:O) SE_AN3.13(D:I1)
N$8: SE_JK4.15(B:Q) SE_JK5.6(A:J) SE_JK9.6(A:J)
N$9: SE_JK4.14(B:!Q) SE_JK5.5(A:K) SE_JK9.5(A:K)
N$10: SE_JK9.10(B:J)
N$11: SE_JK5.2(A:!Q) SE_JK5.11(B:K) SE_JK9.11(B:K)
N$12: SE_JK5.1(A:Q) SE_JK5.10(B:J)
N$13: SE_JK5.15(B:Q) SE_JK6.6(A:J) SE_JK10.6(A:J)
N$14: SE_AN1.2(A:I1) SE_JK8.1(A:Q)
N$15: SE_JK3.15(B:Q) SE_JK4.6(A:J) SE_JK8.6(A:J)
N$16: SE_JK5.14(B:!Q) SE_JK6.5(A:K) SE_JK10.5(A:K)
N$17: SE_JK6.1(A:Q) SE_JK6.10(B:J) SE_JK10.10(B:J)
N$18: SE_JK6.14(B:!Q) SE_JK7.5(A:K) SE_JK11.5(A:K)
N$19: SE_JK7.1(A:Q) SE_JK7.10(B:J) SE_JK11.10(B:J)
N$20: SE_JK6.15(B:Q) SE_JK7.6(A:J) SE_JK11.6(A:J)
N$21: SE_JK7.2(A:!Q) SE_JK7.11(B:K) SE_JK11.11(B:K)
N$22: SE_AN1.1(A:I0) SE_JK8.15(B:Q)
N$23: SE_AN1.9(C:I1) SE_JK9.1(A:Q)
N$24: SE_JK3.14(B:!Q) SE_JK4.5(A:K) SE_JK8.5(A:K)
N$25: SE_JK4.1(A:Q) SE_JK4.10(B:J) SE_JK8.10(B:J)
N$26: SE_JK4.2(A:!Q) SE_JK4.11(B:K) SE_JK8.11(B:K)
N$27: SE_AN1.8(C:I0) SE_JK9.15(B:Q)
N$28: SE_AN1.3(A:O) SE_AN1.6(B:I1)
N$29: SE_JK6.2(A:!Q) SE_JK6.11(B:K) SE_JK10.11(B:K)
N$30: SE_AN1.5(B:I0) SE_AN1.10(C:O)
N$31: SE_AN1.12(D:I0) SE_JK10.15(B:Q)
N$32: SE_AN3.1(A:I0) SE_JK7.15(B:Q)
N$33: SE_AN3.3(A:O) SE_AN3.5(B:I0) SE_JK8.3(A:CLK) SE_JK8.13(B:CLK) SE_JK9.3(A:CLK) SE_JK9.13(B:CLK) SE_JK10.3(A:CLK) SE_JK10.13(B:CLK) SE_JK11.3(A:CLK) SE_JK11.13(B:CLK)
N$34: SE_AN1.4(B:O) SE_AN2.2(A:I1)
N$35: SE_AN1.11(D:O) SE_AN2.1(A:I0)
N$36: SE_JK12.3(A:CLK) SE_JK12.15(B:Q)
N$37: SE_JK1.4(A:R) SE_JK12.4(A:R) SE_JK12.12(B:R) SE_N01.4(B:O)
N$38: M_OR1.2(A:I1) SE_JK1.14(B:!Q) SE_JK2.5(A:K)
N$39: SE_AN3.8(C:I0) SE_JK2.1(A:Q)
N$41: SE_AN3.11(D:O) SE_JK1.13(B:CLK) SE_JK2.3(A:CLK)
N$42: M_OR1.1(A:I0) SE_JK2.2(A:!Q)
N$43: SE_AN2.5(B:I0) SE_JK11.15(B:Q)
N$44: SE_AN2.9(C:I1) SE_JK11.1(A:Q)
N$45: PC_AN5.2(A:I1) SE_AN2.3(A:O) SE_AN2.13(D:I1)
N$46: SE_AN2.10(C:O) SE_AN2.12(D:I0)
N$47: SE_AN2.11(D:O) SE_JK2.9(B:S) SE_N01.7(C:I)
N$48: PC_AN5.1(A:I0) SE_AN2.4(B:O)
N$49: PC_AN5.3(A:O) SE_JK2.12(B:R)
N$153: PC_AN4.1(A:I0) SE_N01.6(C:O)
N$167: PC_AN4.2(A:I1) SE_JK2.15(B:Q)
N$169: SE_BF7.4(Y) SEN7.1
N$170: SE_BF6.4(Y) SEN6.1
N$171: SE_BF5.4(Y) SEN5.1
N$172: SE_BF4.4(Y) SEN4.2
N$173: SE_BF3.4(Y) SEN3.2
N$174: SE_BF2.4(Y) SEN2.2
N$175: SE_BF1.4(Y) SEN1.2
N$176: SE_BF0.4(Y) SEN0.2
N$178: SE_CLK.1 SE_JK12.1(A:Q)
N$200: SE_AN2.8(C:I0) SE_BF7.2(A) SE_JK11.14(B:!Q)
N$201: SE_AN2.6(B:I1) SE_BF6.2(A) SE_JK11.2(A:!Q)
N$202: SE_BF5.2(A) SE_JK10.14(B:!Q)
N$203: SE_AN1.13(D:I1) SE_BF4.2(A) SE_JK10.2(A:!Q)
N$204: SE_BF3.2(A) SE_JK9.14(B:!Q)
N$205: SE_BF0.2(A) SE_JK8.2(A:!Q)
N$206: SE_BF1.2(A) SE_JK8.14(B:!Q)
N$207: SE_BF2.2(A) SE_JK9.2(A:!Q)
SE_CLK: SE_AN3.6(B:I1) SE_CLK.2 SE_JK3.3(A:CLK) SE_JK3.13(B:CLK) SE_JK4.3(A:CLK) SE_JK4.13(B:CLK) SE_JK5.3(A:CLK) SE_JK5.13(B:CLK) SE_JK6.3(A:CLK) SE_JK6.13(B:CLK) SE_JK7.3(A:CLK) SE_JK7.13(B:CLK)
SE_ENCLK: SE_AN3.10(C:O) SE_JK1.5(A:K) SE_JK1.6(A:J) SE_JK12.5(A:K) SE_JK12.6(A:J) SE_JK12.10(B:J) SE_JK12.11(B:K) SE_N01.5(B:I)
SE_N0: SEN0.1 ; also sheet 5
SE_N1: SEN1.1 ; also sheet 5
SE_N2: SEN2.1 ; also sheet 5
SE_N3: SEN3.1 ; also sheet 5
SE_N4: SEN4.1 ; also sheet 5
SE_N5: SEN5.2 ; also sheet 5
SE_N6: SEN6.2 ; also sheet 5
SE_N7: SEN7.2 ; also sheet 5
SE_NEWNUMBER: SE_AN3.4(B:O) SE_JK1.12(B:R) SE_JK2.4(A:R) SE_JK3.4(A:R) SE_JK3.12(B:R) SE_JK4.4(A:R) SE_JK4.12(B:R) SE_JK5.4(A:R) SE_JK5.12(B:R) SE_JK6.4(A:R) SE_JK6.12(B:R) SE_JK7.4(A:R) SE_JK7.12(B:R) ; also sheet 2
SE_WRITE_N: SE_JK2.14(B:!Q) ; also sheet 1,2,5
SE_WRITE_P: PC_AN4.3(A:O) SE_BF0.1(OE) SE_BF1.1(OE) SE_BF2.1(OE) SE_BF3.1(OE) SE_BF4.1(OE) SE_BF5.1(OE) SE_BF6.1(OE) SE_BF7.1(OE) ; also sheet 1,2,5
Unconnected: BR_NO1.3(A:I) FT232.2(DTR) FT232.3(RTS) FT232.5(RXD) FT232.6(RI) FT232.9(DSR) FT232.10(DCD) FT232.11(CTS) FT232.12(CBUS4) FT232.13(CBUS2) FT232.14(CBUS3) FT232.17(3V3OUT) FT232.22(CBUS1) FT232.23(CBUS0) FT232.27(OSCIN) FT232.28(OSCOUT) PC_NO1.3(A:I) PC_NO1.5(B:I) SE_JK1.2(A:!Q) SE_JK2.10(B:J) SE_JK2.11(B:K) SE_JK2.13(B:CLK) SE_JK7.14(B:!Q) SE_JK10.1(A:Q) SE_JK12.2(A:!Q) SE_JK12.14(B:!Q) SE_N01.9(D:I) SE_N01.11(E:I) SE_N01.14(F:I)

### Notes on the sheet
- SE=Serielle
- Sie liest die Serielle aus und gibt 10 bit zurück: 
  8 bit Daten
  1 bit um sie zu speichern wird bei 0000 1001 auf HIGH und bei 0000 1010 auf LOW gesetzt
  1 bit um eine neue Zahl anzuzeigen
  
  braucht 3 bit daten
  1 bit M_CLK ist die clock
  2 bit Serieller Input
- Dieser Teil sorgt dafür, dass nur wenn das startbyte 
  gelesen wurde, die Daten durchkommen
- Dieser Teil ist ein einfaches schiebe register, dass das Signal einfach nacheinander weiterschiebt. | Most Significant bit
- 0 1010 1010 1
- Dieser Teil invertiert zuerst das Signal und wartet bis beide 
  jk flipflops HIGH sind, um beim Auslesen ungefähr in der Mitte zu treffen.
- Dieser Teil erkennt wenn am Ende des 
  Schieberegisters eine 1 und
  am Anfang eine 0 ist, wenn es stimmt 
  wird die clock weiter gegeben. 
  0 xxxx xxxx 1
- Dieser Teil speichert bei HIGH das im Schieberegister 
  befindene Byte ohne dem Stop und Start bit ab
- Dieser Teil wandelt mit Hilfe von einem FT232 ein
  RS232 USB Daten in eine Serielle um und gibt sie aus.
- Dieser Teil nimmt die Main clock die 1200 Hz beträgt und
  wandelt sie bei HIGH in 300Hz welches dann weiter verwendet wird.
- wenn eine Nummer eingelesen wurde wird SE_NEWNUMBER kurzzeitig HIGH
- 0000 1001
- Dieser Teil erkennt eine bestimmte bytekombination die aussagt ob der Speicher beschrieben werden soll oder nicht und
  deswegen muss vor dem Senden der Daten zuerst 0000 1001 gesendet werden damit die darauffolgende Daten im Sytem und in den Speicher gelangen
- SE_WRITE 
  0000 1001 HIGH
  0000 1010 LOW
- 0000 1010
- Least Significant bit

## Sheet 4 of 5: JMP/bra
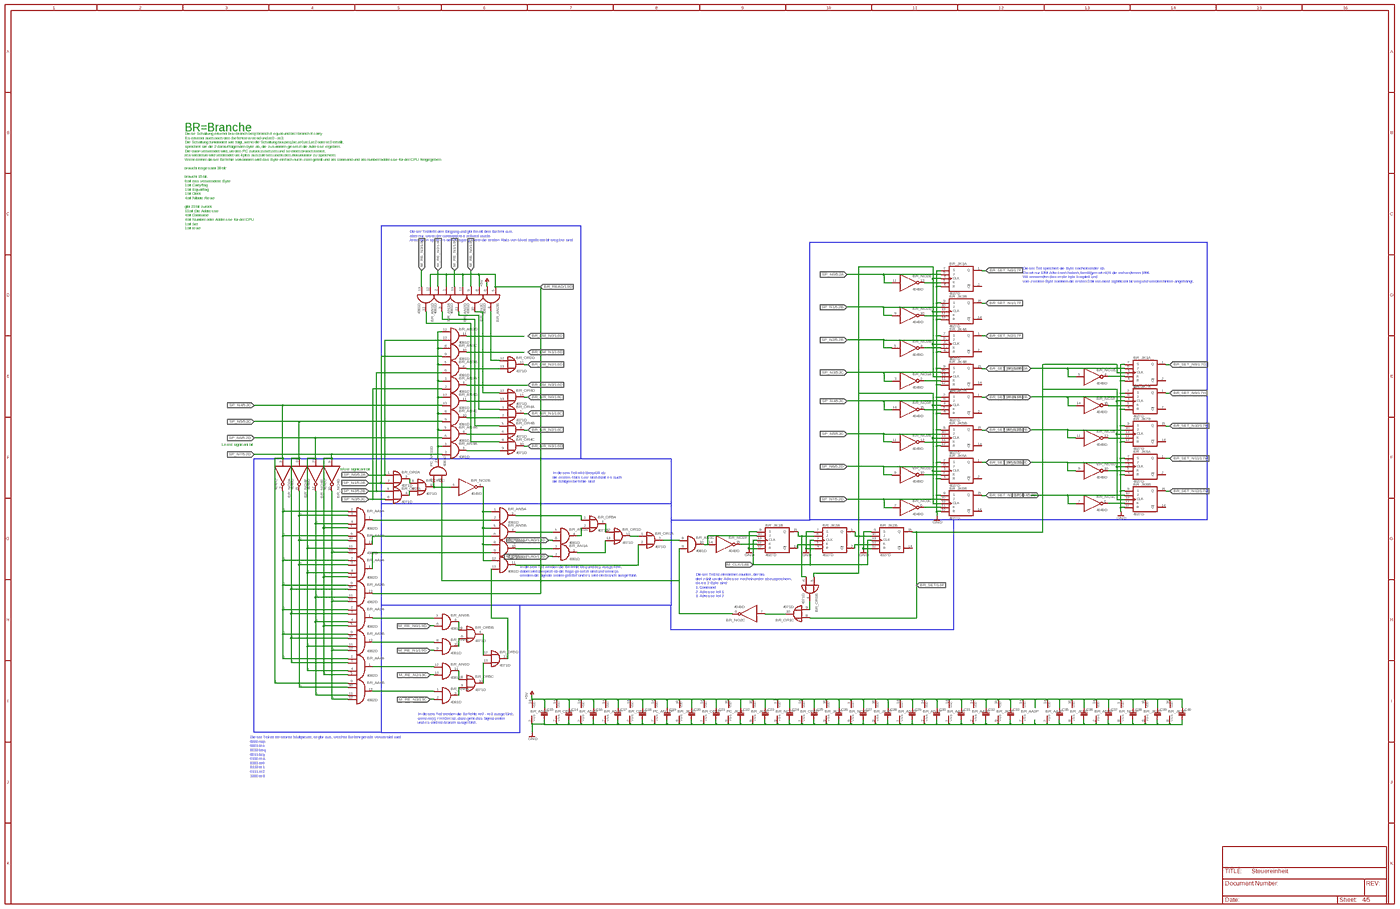
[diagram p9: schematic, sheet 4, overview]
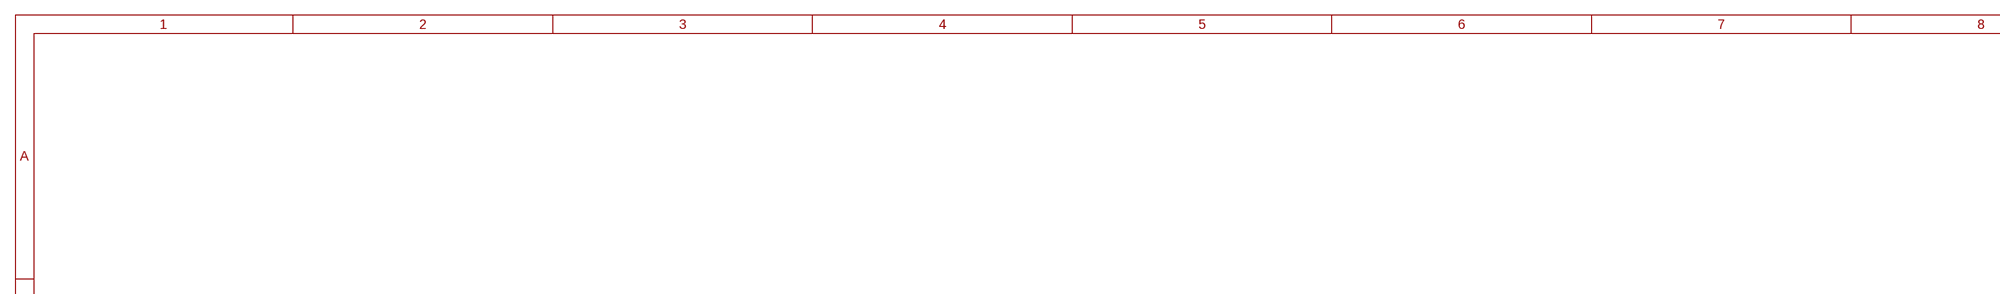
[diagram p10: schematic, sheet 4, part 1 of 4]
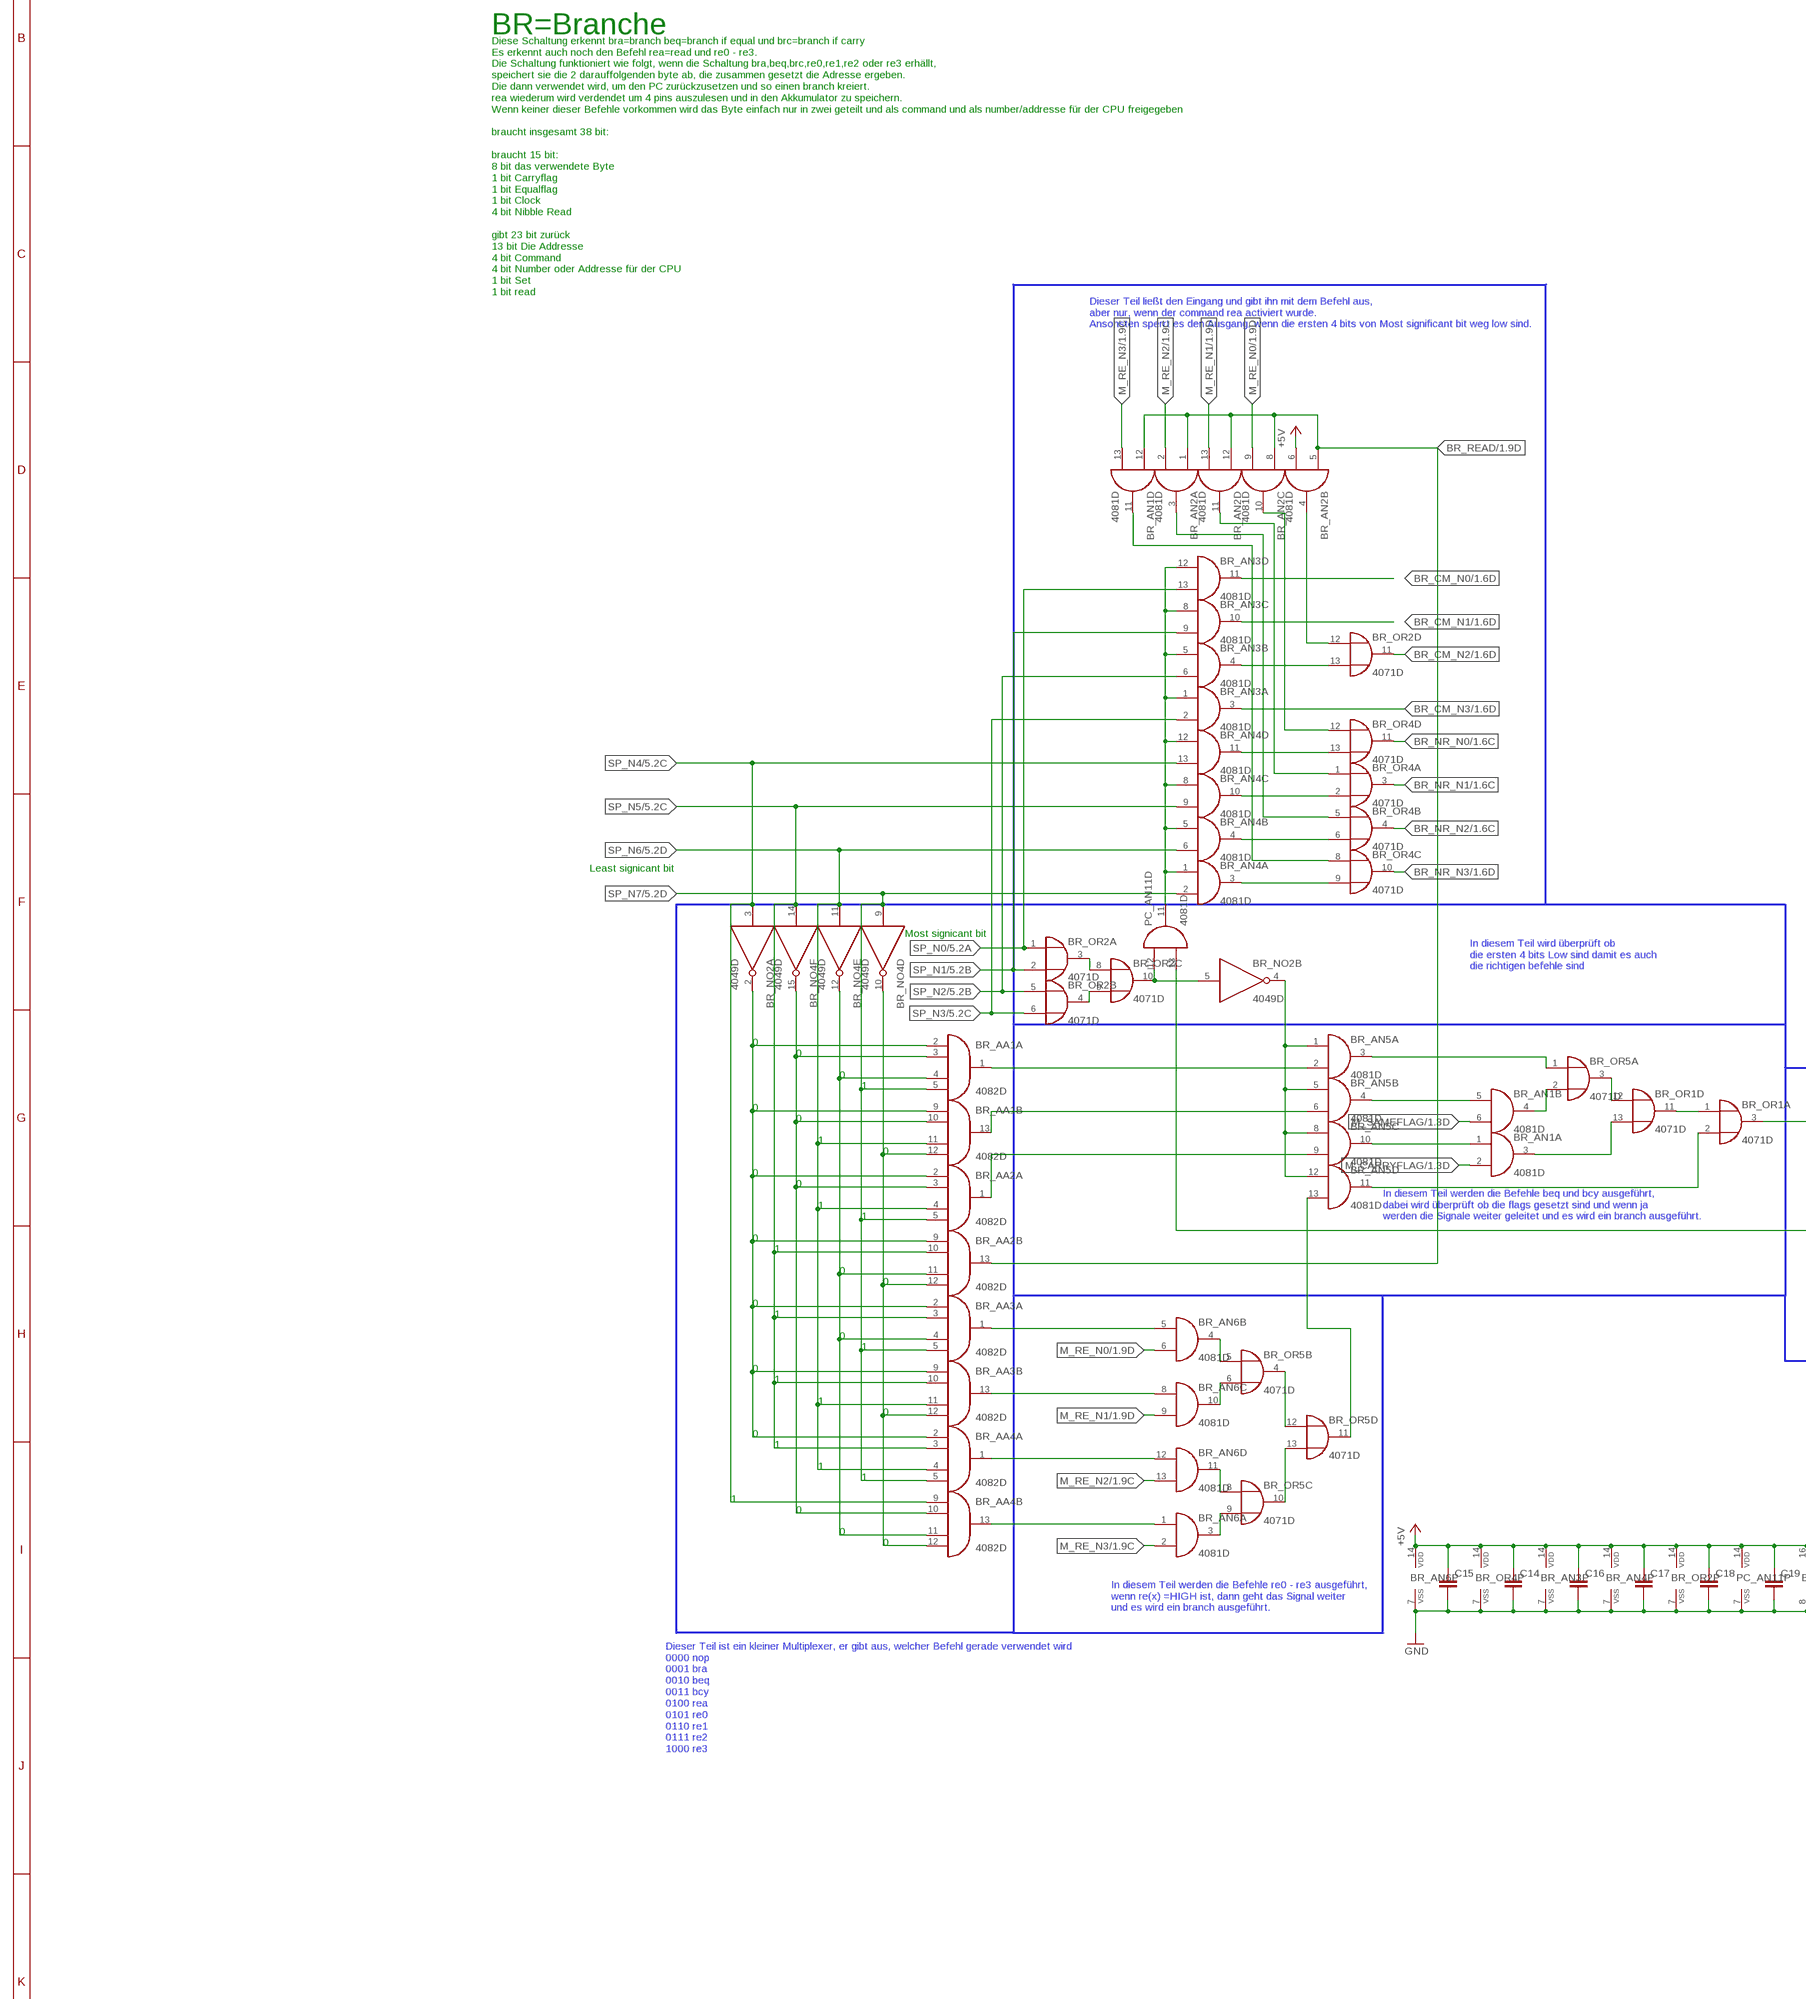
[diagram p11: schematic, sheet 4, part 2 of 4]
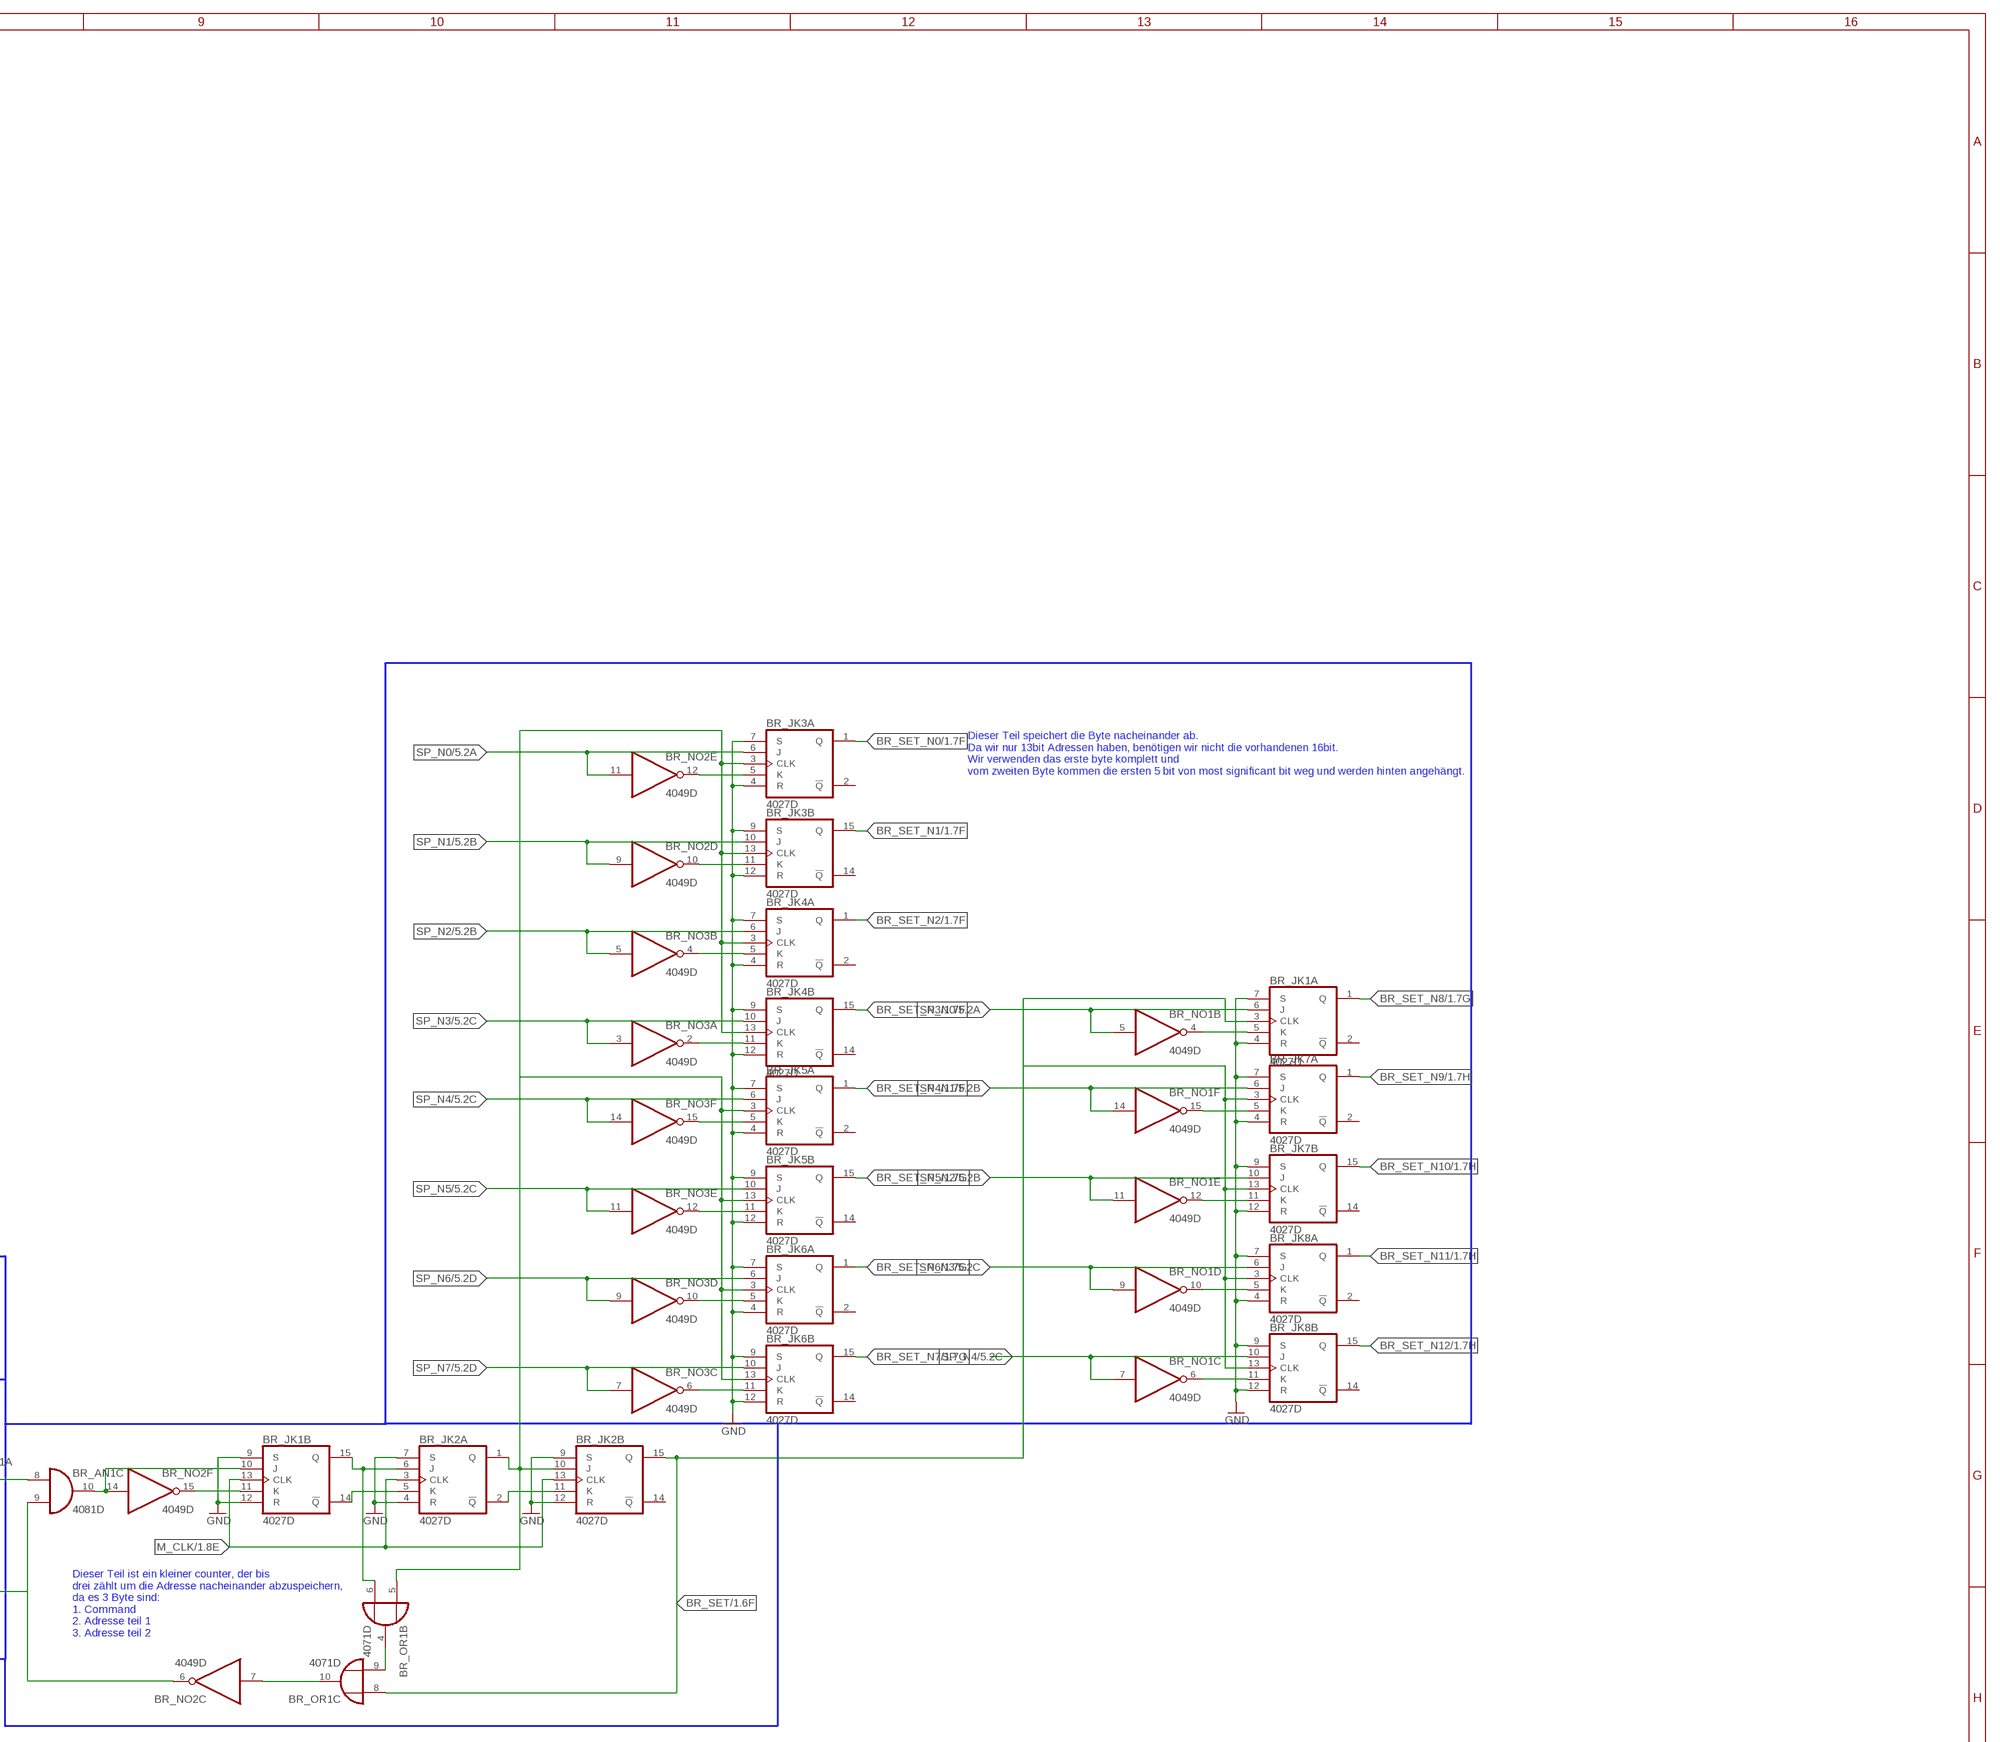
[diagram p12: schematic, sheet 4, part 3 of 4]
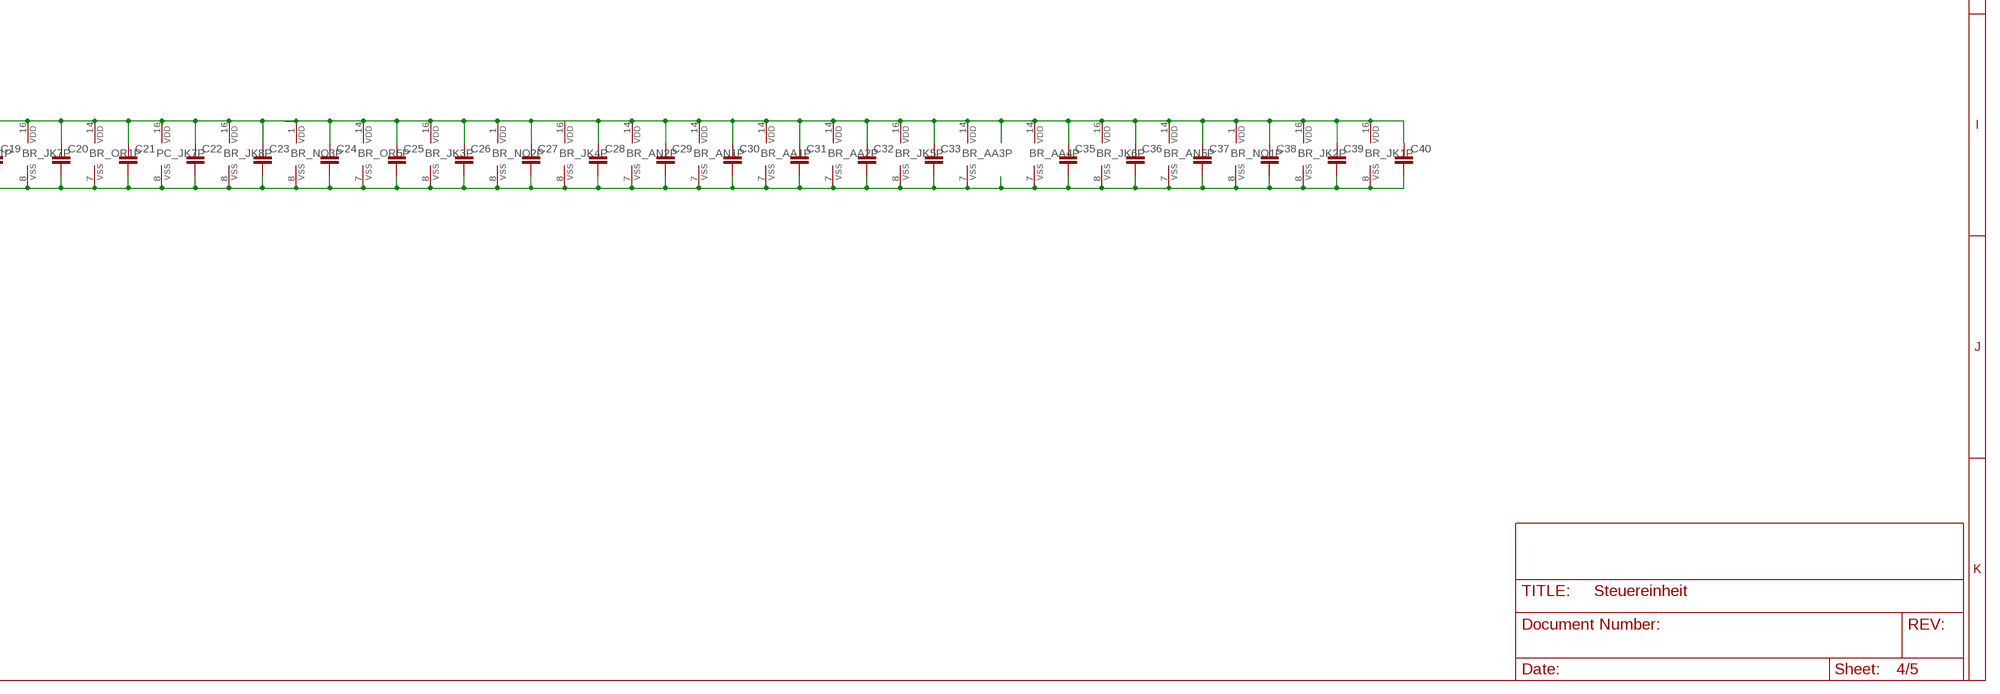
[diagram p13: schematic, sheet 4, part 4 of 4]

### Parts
BR_AA1  4082D  [SO14]
BR_AA2  4082D  [SO14]
BR_AA3  4082D  [SO14]
BR_AA4  4082D  [SO14]
BR_AN1  4081D  [SO14]
BR_AN2  4081D  [SO14]
BR_AN3  4081D  [SO14]
BR_AN4  4081D  [SO14]
BR_AN5  4081D  [SO14]
BR_AN6  4081D  [SO14]
BR_JK1  4027D  [SO16]
BR_JK2  4027D  [SO16]
BR_JK3  4027D  [SO16]
BR_JK4  4027D  [SO16]
BR_JK5  4027D  [SO16]
BR_JK6  4027D  [SO16]
BR_JK7  4027D  [SO16]
BR_JK8  4027D  [SO16]
BR_NO2  4049D  [SO16]
BR_NO3  4049D  [SO16]
BR_OR1  4071D  [SO14]
BR_OR2  4071D  [SO14]
BR_OR4  4071D  [SO14]
BR_OR5  4071D  [SO14]
C14  C-EUC0805  [C0805]
C15  C-EUC0805  [C0805]
C16  C-EUC0805  [C0805]
C17  C-EUC0805  [C0805]
C18  C-EUC0805  [C0805]
C19  C-EUC0805  [C0805]
C20  C-EUC0805  [C0805]
C21  C-EUC0805  [C0805]
C22  C-EUC0805  [C0805]
C23  C-EUC0805  [C0805]
C24  C-EUC0805  [C0805]
C25  C-EUC0805  [C0805]
C26  C-EUC0805  [C0805]
C27  C-EUC0805  [C0805]
C28  C-EUC0805  [C0805]
C29  C-EUC0805  [C0805]
C30  C-EUC0805  [C0805]
C31  C-EUC0805  [C0805]
C32  C-EUC0805  [C0805]
C33  C-EUC0805  [C0805]
C35  C-EUC0805  [C0805]
C36  C-EUC0805  [C0805]
C37  C-EUC0805  [C0805]
C38  C-EUC0805  [C0805]
C39  C-EUC0805  [C0805]
C40  C-EUC0805  [C0805]

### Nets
+5V: BR_AA1.14(P:VDD) BR_AA2.14(P:VDD) BR_AA3.14(P:VDD) BR_AA4.14(P:VDD) BR_AN1.14(P:VDD) BR_AN2.6(B:I1) BR_AN2.14(P:VDD) BR_AN3.14(P:VDD) BR_AN4.14(P:VDD) BR_AN5.14(P:VDD) BR_AN6.14(P:VDD) BR_JK1.16(P:VDD) BR_JK2.16(P:VDD) BR_JK3.16(P:VDD) BR_JK4.16(P:VDD) BR_JK5.16(P:VDD) BR_JK6.16(P:VDD) BR_JK7.16(P:VDD) BR_JK8.16(P:VDD) BR_NO1.1(P:VDD) BR_NO2.1(P:VDD) BR_NO3.1(P:VDD) BR_OR1.14(P:VDD) BR_OR2.14(P:VDD) BR_OR4.14(P:VDD) BR_OR5.14(P:VDD) C14.1 C15.1 C16.1 C17.1 C18.1 C19.1 C20.1 C21.1 C22.1 C23.1 C24.1 C25.1 C26.1 C27.1 C28.1 C29.1 C30.1 C31.1 C32.1 C33.1 C35.1 C36.1 C37.1 C38.1 C39.1 C40.1 PC_AN11.14(P:VDD) PC_JK7.16(P:VDD) ; also sheet 1,2,3,5
BR_CM_N0: BR_AN3.11(D:O) ; also sheet 1
BR_CM_N1: BR_AN3.10(C:O) ; also sheet 1
BR_CM_N2: BR_OR2.11(D:O) ; also sheet 1
BR_CM_N3: BR_AN3.3(A:O) ; also sheet 1
BR_NR_N0: BR_OR4.11(D:O) ; also sheet 1
BR_NR_N1: BR_OR4.3(A:O) ; also sheet 1
BR_NR_N2: BR_OR4.4(B:O) ; also sheet 1
BR_NR_N3: BR_OR4.10(C:O) ; also sheet 1
BR_READ: BR_AA2.13(B:O) BR_AN1.12(D:I0) BR_AN2.1(A:I0) BR_AN2.5(B:I0) BR_AN2.8(C:I0) BR_AN2.12(D:I0) ; also sheet 1
BR_SET: BR_JK2.15(B:Q) BR_JK7.3(A:CLK) BR_JK7.13(B:CLK) BR_JK8.3(A:CLK) BR_JK8.13(B:CLK) BR_OR1.8(C:I0) ; also sheet 1
BR_SET_N0: BR_JK3.1(A:Q) ; also sheet 1
BR_SET_N1: BR_JK3.15(B:Q) ; also sheet 1
BR_SET_N2: BR_JK4.1(A:Q) ; also sheet 1
BR_SET_N3: BR_JK4.15(B:Q) ; also sheet 1
BR_SET_N4: BR_JK5.1(A:Q) ; also sheet 1
BR_SET_N5: BR_JK5.15(B:Q) ; also sheet 1
BR_SET_N6: BR_JK6.1(A:Q) ; also sheet 1
BR_SET_N7: BR_JK6.15(B:Q) ; also sheet 1
BR_SET_N8: BR_JK1.1(A:Q) ; also sheet 1
BR_SET_N9: BR_JK7.1(A:Q) ; also sheet 1
BR_SET_N10: BR_JK7.15(B:Q) ; also sheet 1
BR_SET_N11: BR_JK8.1(A:Q) ; also sheet 1
BR_SET_N12: BR_JK8.15(B:Q) ; also sheet 1
GND: BR_AA1.7(P:VSS) BR_AA2.7(P:VSS) BR_AA3.7(P:VSS) BR_AA4.7(P:VSS) BR_AN1.7(P:VSS) BR_AN2.7(P:VSS) BR_AN3.7(P:VSS) BR_AN4.7(P:VSS) BR_AN5.7(P:VSS) BR_AN6.7(P:VSS) BR_JK1.8(P:VSS) BR_JK1.9(B:S) BR_JK1.12(B:R) BR_JK2.4(A:R) BR_JK2.7(A:S) BR_JK2.8(P:VSS) BR_JK2.9(B:S) BR_JK2.12(B:R) BR_JK3.4(A:R) BR_JK3.7(A:S) BR_JK3.8(P:VSS) BR_JK3.9(B:S) BR_JK3.12(B:R) BR_JK4.4(A:R) BR_JK4.7(A:S) BR_JK4.8(P:VSS) BR_JK4.9(B:S) BR_JK4.12(B:R) BR_JK5.4(A:R) BR_JK5.7(A:S) BR_JK5.8(P:VSS) BR_JK5.9(B:S) BR_JK5.12(B:R) BR_JK6.4(A:R) BR_JK6.7(A:S) BR_JK6.8(P:VSS) BR_JK6.9(B:S) BR_JK6.12(B:R) BR_JK7.4(A:R) BR_JK7.7(A:S) BR_JK7.8(P:VSS) BR_JK7.9(B:S) BR_JK7.12(B:R) BR_JK8.4(A:R) BR_JK8.7(A:S) BR_JK8.8(P:VSS) BR_JK8.9(B:S) BR_JK8.12(B:R) BR_NO1.8(P:VSS) BR_NO2.8(P:VSS) BR_NO3.8(P:VSS) BR_OR1.7(P:VSS) BR_OR2.7(P:VSS) BR_OR4.7(P:VSS) BR_OR5.7(P:VSS) C14.2 C15.2 C16.2 C17.2 C18.2 C19.2 C20.2 C21.2 C22.2 C23.2 C24.2 C25.2 C26.2 C27.2 C28.2 C29.2 C30.2 C31.2 C32.2 C33.2 C35.2 C36.2 C37.2 C38.2 C39.2 C40.2 PC_AN11.7(P:VSS) PC_JK7.8(P:VSS) ; also sheet 1,2,3,5
GND2: BR_JK1.4(A:R) BR_JK1.7(A:S)
M_CARRYFLAG: BR_AN1.2(A:I1) ; also sheet 1
M_CLK: BR_JK1.13(B:CLK) BR_JK2.3(A:CLK) BR_JK2.13(B:CLK) ; also sheet 1,2,3
M_RE_N0: BR_AN2.9(C:I1) BR_AN6.6(B:I1) ; also sheet 1
M_RE_N1: BR_AN2.13(D:I1) BR_AN6.9(C:I1) ; also sheet 1
M_RE_N2: BR_AN2.2(A:I1) BR_AN6.13(D:I1) ; also sheet 1
M_RE_N3: BR_AN1.13(D:I1) BR_AN6.2(A:I1) ; also sheet 1
M_SAMEFLAG: BR_AN1.6(B:I1) ; also sheet 1
N$61: BR_NO2.5(B:I) BR_OR2.10(C:O) PC_AN11.12(D:I0)
N$89: BR_AN1.10(C:O) BR_JK1.10(B:J) BR_NO2.14(F:I)
N$90: BR_OR2.4(B:O) BR_OR2.9(C:I1)
N$92: BR_OR2.3(A:O) BR_OR2.8(C:I0)
N$94: BR_AN1.8(C:I0) BR_OR1.3(A:O)
N$96: BR_AN3.4(B:O) BR_OR2.13(D:I1)
N$98: BR_JK1.11(B:K) BR_NO2.15(F:O)
N$100: BR_AN3.1(A:I0) BR_AN3.5(B:I0) BR_AN3.8(C:I0) BR_AN3.12(D:I0) BR_AN4.1(A:I0) BR_AN4.5(B:I0) BR_AN4.8(C:I0) BR_AN4.12(D:I0) PC_AN11.11(D:O)
N$102: BR_AN4.11(D:O) BR_OR4.13(D:I1)
N$104: BR_AN4.10(C:O) BR_OR4.2(A:I1)
N$106: BR_AN4.4(B:O) BR_OR4.6(B:I1)
N$108: BR_AN4.3(A:O) BR_OR4.9(C:I1)
N$110: BR_JK6.11(B:K) BR_NO3.6(C:O)
N$112: BR_OR1.4(B:O) BR_OR1.9(C:I1)
N$114: BR_AN2.4(B:O) BR_OR2.12(D:I0)
N$115: BR_JK3.3(A:CLK) BR_JK3.13(B:CLK) BR_JK4.3(A:CLK) BR_JK4.13(B:CLK)
N$116: BR_AN2.10(C:O) BR_OR4.12(D:I0)
N$117: BR_AN2.11(D:O) BR_OR4.1(A:I0)
N$118: BR_AN2.3(A:O) BR_OR4.5(B:I0)
N$119: BR_AN1.11(D:O) BR_OR4.8(C:I0)
N$120: BR_AA1.12(B:I3) BR_AA2.12(B:I3) BR_AA3.12(B:I3) BR_AA4.12(B:I3) BR_NO4.10(D:O)
N$121: BR_AA1.4(A:I2) BR_AA2.11(B:I2) BR_AA3.4(A:I2) BR_AA4.11(B:I2) BR_NO4.12(E:O)
N$122: BR_AA1.3(A:I1) BR_AA1.10(B:I1) BR_AA2.3(A:I1) BR_AA4.10(B:I1) BR_NO4.15(F:O)
N$123: BR_AA1.2(A:I0) BR_AA1.9(B:I0) BR_AA2.2(A:I0) BR_AA2.9(B:I0) BR_AA3.2(A:I0) BR_AA3.9(B:I0) BR_AA4.2(A:I0) BR_NO2.2(A:O)
N$124: BR_JK6.5(A:K) BR_NO3.10(D:O)
N$125: BR_AA1.1(A:O) BR_AN5.2(A:I1)
N$126: BR_AA1.13(B:O) BR_AN5.6(B:I1)
N$127: BR_AN5.1(A:I0) BR_AN5.5(B:I0) BR_AN5.8(C:I0) BR_AN5.12(D:I0) BR_NO2.4(B:O)
N$128: BR_AN1.5(B:I0) BR_AN5.4(B:O)
N$129: BR_AN5.3(A:O) BR_OR5.1(A:I0)
N$130: BR_AN1.4(B:O) BR_OR5.2(A:I1)
N$131: BR_AA2.1(A:O) BR_AN5.9(C:I1)
N$132: BR_AN1.1(A:I0) BR_AN5.10(C:O)
N$133: BR_AN1.3(A:O) BR_OR1.13(D:I1)
N$134: BR_OR1.12(D:I0) BR_OR5.3(A:O)
N$135: BR_AA3.1(A:O) BR_AN6.5(B:I0)
N$136: BR_AA3.13(B:O) BR_AN6.8(C:I0)
N$137: BR_AA4.1(A:O) BR_AN6.12(D:I0)
N$138: BR_AA4.13(B:O) BR_AN6.1(A:I0)
N$139: BR_AN6.4(B:O) BR_OR5.5(B:I0)
N$140: BR_AN6.10(C:O) BR_OR5.6(B:I1)
N$141: BR_OR5.4(B:O) BR_OR5.12(D:I0)
N$142: BR_OR5.10(C:O) BR_OR5.13(D:I1)
N$143: BR_AN6.11(D:O) BR_OR5.8(C:I0)
N$144: BR_AN6.3(A:O) BR_OR5.9(C:I1)
N$145: BR_AN5.13(D:I1) BR_OR5.11(D:O)
N$146: BR_AN5.11(D:O) BR_OR1.2(A:I1)
N$147: BR_OR1.1(A:I0) BR_OR1.11(D:O)
N$148: BR_JK1.14(B:!Q) BR_JK2.5(A:K)
N$149: BR_JK5.11(B:K) BR_NO3.12(E:O)
N$150: BR_JK2.1(A:Q) BR_JK2.10(B:J) BR_JK5.3(A:CLK) BR_JK5.13(B:CLK) BR_JK6.3(A:CLK) BR_JK6.13(B:CLK) BR_OR1.5(B:I0)
N$151: BR_JK2.2(A:!Q) BR_JK2.11(B:K)
N$152: BR_JK5.5(A:K) BR_NO3.15(F:O)
N$154: BR_AN1.9(C:I1) BR_NO2.6(C:O) PC_AN11.13(D:I1)
N$155: BR_NO2.7(C:I) BR_OR1.10(C:O)
N$156: BR_JK8.11(B:K) BR_NO1.6(C:O)
N$157: BR_JK8.5(A:K) BR_NO1.10(D:O)
N$158: BR_JK7.11(B:K) BR_NO1.12(E:O)
N$159: BR_JK1.15(B:Q) BR_JK2.6(A:J) BR_OR1.6(B:I1)
N$160: BR_JK4.11(B:K) BR_NO3.2(A:O)
N$161: BR_JK4.5(A:K) BR_NO3.4(B:O)
N$162: BR_JK3.11(B:K) BR_NO2.10(D:O)
N$163: BR_JK3.5(A:K) BR_NO2.12(E:O)
N$164: BR_JK7.5(A:K) BR_NO1.15(F:O)
N$165: BR_JK1.3(A:CLK)
N$166: BR_JK1.5(A:K) BR_NO1.4(B:O)
SP_N0: BR_AN3.13(D:I1) BR_JK1.6(A:J) BR_JK3.6(A:J) BR_NO1.5(B:I) BR_NO2.11(E:I) BR_OR2.1(A:I0) ; also sheet 5
SP_N1: BR_AN3.9(C:I1) BR_JK3.10(B:J) BR_JK7.6(A:J) BR_NO1.14(F:I) BR_NO2.9(D:I) BR_OR2.2(A:I1) ; also sheet 5
SP_N2: BR_AN3.6(B:I1) BR_JK4.6(A:J) BR_JK7.10(B:J) BR_NO1.11(E:I) BR_NO3.5(B:I) BR_OR2.5(B:I0) ; also sheet 5
SP_N3: BR_AN3.2(A:I1) BR_JK4.10(B:J) BR_JK8.6(A:J) BR_NO1.9(D:I) BR_NO3.3(A:I) BR_OR2.6(B:I1) ; also sheet 5
SP_N4: BR_AA4.9(B:I0) BR_AN4.13(D:I1) BR_JK5.6(A:J) BR_JK8.10(B:J) BR_NO1.7(C:I) BR_NO2.3(A:I) BR_NO3.14(F:I) ; also sheet 5
SP_N5: BR_AA2.10(B:I1) BR_AA3.3(A:I1) BR_AA3.10(B:I1) BR_AA4.3(A:I1) BR_AN4.9(C:I1) BR_JK5.10(B:J) BR_NO3.11(E:I) BR_NO4.14(F:I) ; also sheet 5
SP_N6: BR_AA1.11(B:I2) BR_AA2.4(A:I2) BR_AA3.11(B:I2) BR_AA4.4(A:I2) BR_AN4.6(B:I1) BR_JK6.6(A:J) BR_NO3.9(D:I) BR_NO4.11(E:I) ; also sheet 5
SP_N7: BR_AA1.5(A:I3) BR_AA2.5(A:I3) BR_AA3.5(A:I3) BR_AA4.5(A:I3) BR_AN4.2(A:I1) BR_JK6.10(B:J) BR_NO3.7(C:I) BR_NO4.9(D:I) ; also sheet 5
Unconnected: BR_JK1.2(A:!Q) BR_JK2.14(B:!Q) BR_JK3.2(A:!Q) BR_JK3.14(B:!Q) BR_JK4.2(A:!Q) BR_JK4.14(B:!Q) BR_JK5.2(A:!Q) BR_JK5.14(B:!Q) BR_JK6.2(A:!Q) BR_JK6.14(B:!Q) BR_JK7.2(A:!Q) BR_JK7.14(B:!Q) BR_JK8.2(A:!Q) BR_JK8.14(B:!Q)

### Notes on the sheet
- BR=Branche
- Diese Schaltung erkennt bra=branch beq=branch if equal und brc=branch if carry
  Es erkennt auch noch den Befehl rea=read und re0 - re3.
  Die Schaltung funktioniert wie folgt, wenn die Schaltung bra,beq,brc,re0,re1,re2 oder re3 erhällt, 
  speichert sie die 2 darauffolgenden byte ab, die zusammen gesetzt die Adresse ergeben.
  Die dann verwendet wird, um den PC zurückzusetzen und so einen branch kreiert.
  rea wiederum wird verdendet um 4 pins auszulesen und in den Akkumulator zu speichern.
  Wenn keiner dieser Befehle vorkommen wird das Byte einfach nur in zwei geteilt und als command und als number/addresse für der CPU freigegeben
  
  braucht insgesamt 38 bit:
  
  braucht 15 bit:
  8 bit das verwendete Byte
  1 bit Carryflag
  1 bit Equalflag
  1 bit Clock
  4 bit Nibble Read
  
  gibt 23 bit zurück
  13 bit Die Addresse
  4 bit Command
  4 bit Number oder Addresse für der CPU
  1 bit Set
  1 bit read
- Dieser Teil ließt den Eingang und gibt ihn mit dem Befehl aus, 
  aber nur, wenn der command rea activiert wurde.
  Ansonsten sperrt es den Ausgang, wenn die ersten 4 bits von Most significant bit weg low sind.
- Dieser Teil speichert die Byte nacheinander ab.
  Da wir nur 13bit Adressen haben, benötigen wir nicht die vorhandenen 16bit.
  Wir verwenden das erste byte komplett und
  vom zweiten Byte kommen die ersten 5 bit von most significant bit weg und werden hinten angehängt.
- Least signicant bit
- Most signicant bit
- In diesem Teil wird überprüft ob 
  die ersten 4 bits Low sind damit es auch 
  die richtigen befehle sind
- 0
- 0
- 0
- 1
- 0
- 0
- 1
- 0
- 0
- 0
- 1
- 1
- In diesem Teil werden die Befehle beq und bcy ausgeführt,
  dabei wird überprüft ob die flags gesetzt sind und wenn ja
  werden die Signale weiter geleitet und es wird ein branch ausgeführt.
- 0
- 1
- 0
- Dieser Teil ist ein kleiner counter, der bis
  drei zählt um die Adresse nacheinander abzuspeichern,
  da es 3 Byte sind:
  1. Command
  2. Adresse teil 1
  3. Adresse teil 2
- 0
- 0
- 1
- 0
- 1
- 0
- 1
- 1
- 0
- 0
- 1
- 1
- 1
- 1
- 0
- 0
- 0
- In diesem Teil werden die Befehle re0 - re3 ausgeführt,
  wenn re(x) =HIGH ist, dann geht das Signal weiter
  und es wird ein branch ausgeführt.
- Dieser Teil ist ein kleiner Multiplexer, er gibt aus, welcher Befehl gerade verwendet wird
  0000 nop
  0001 bra
  0010 beq
  0011 bcy
  0100 rea
  0101 re0
  0110 re1
  0111 re2
  1000 re3

## Sheet 5 of 5: Speicher
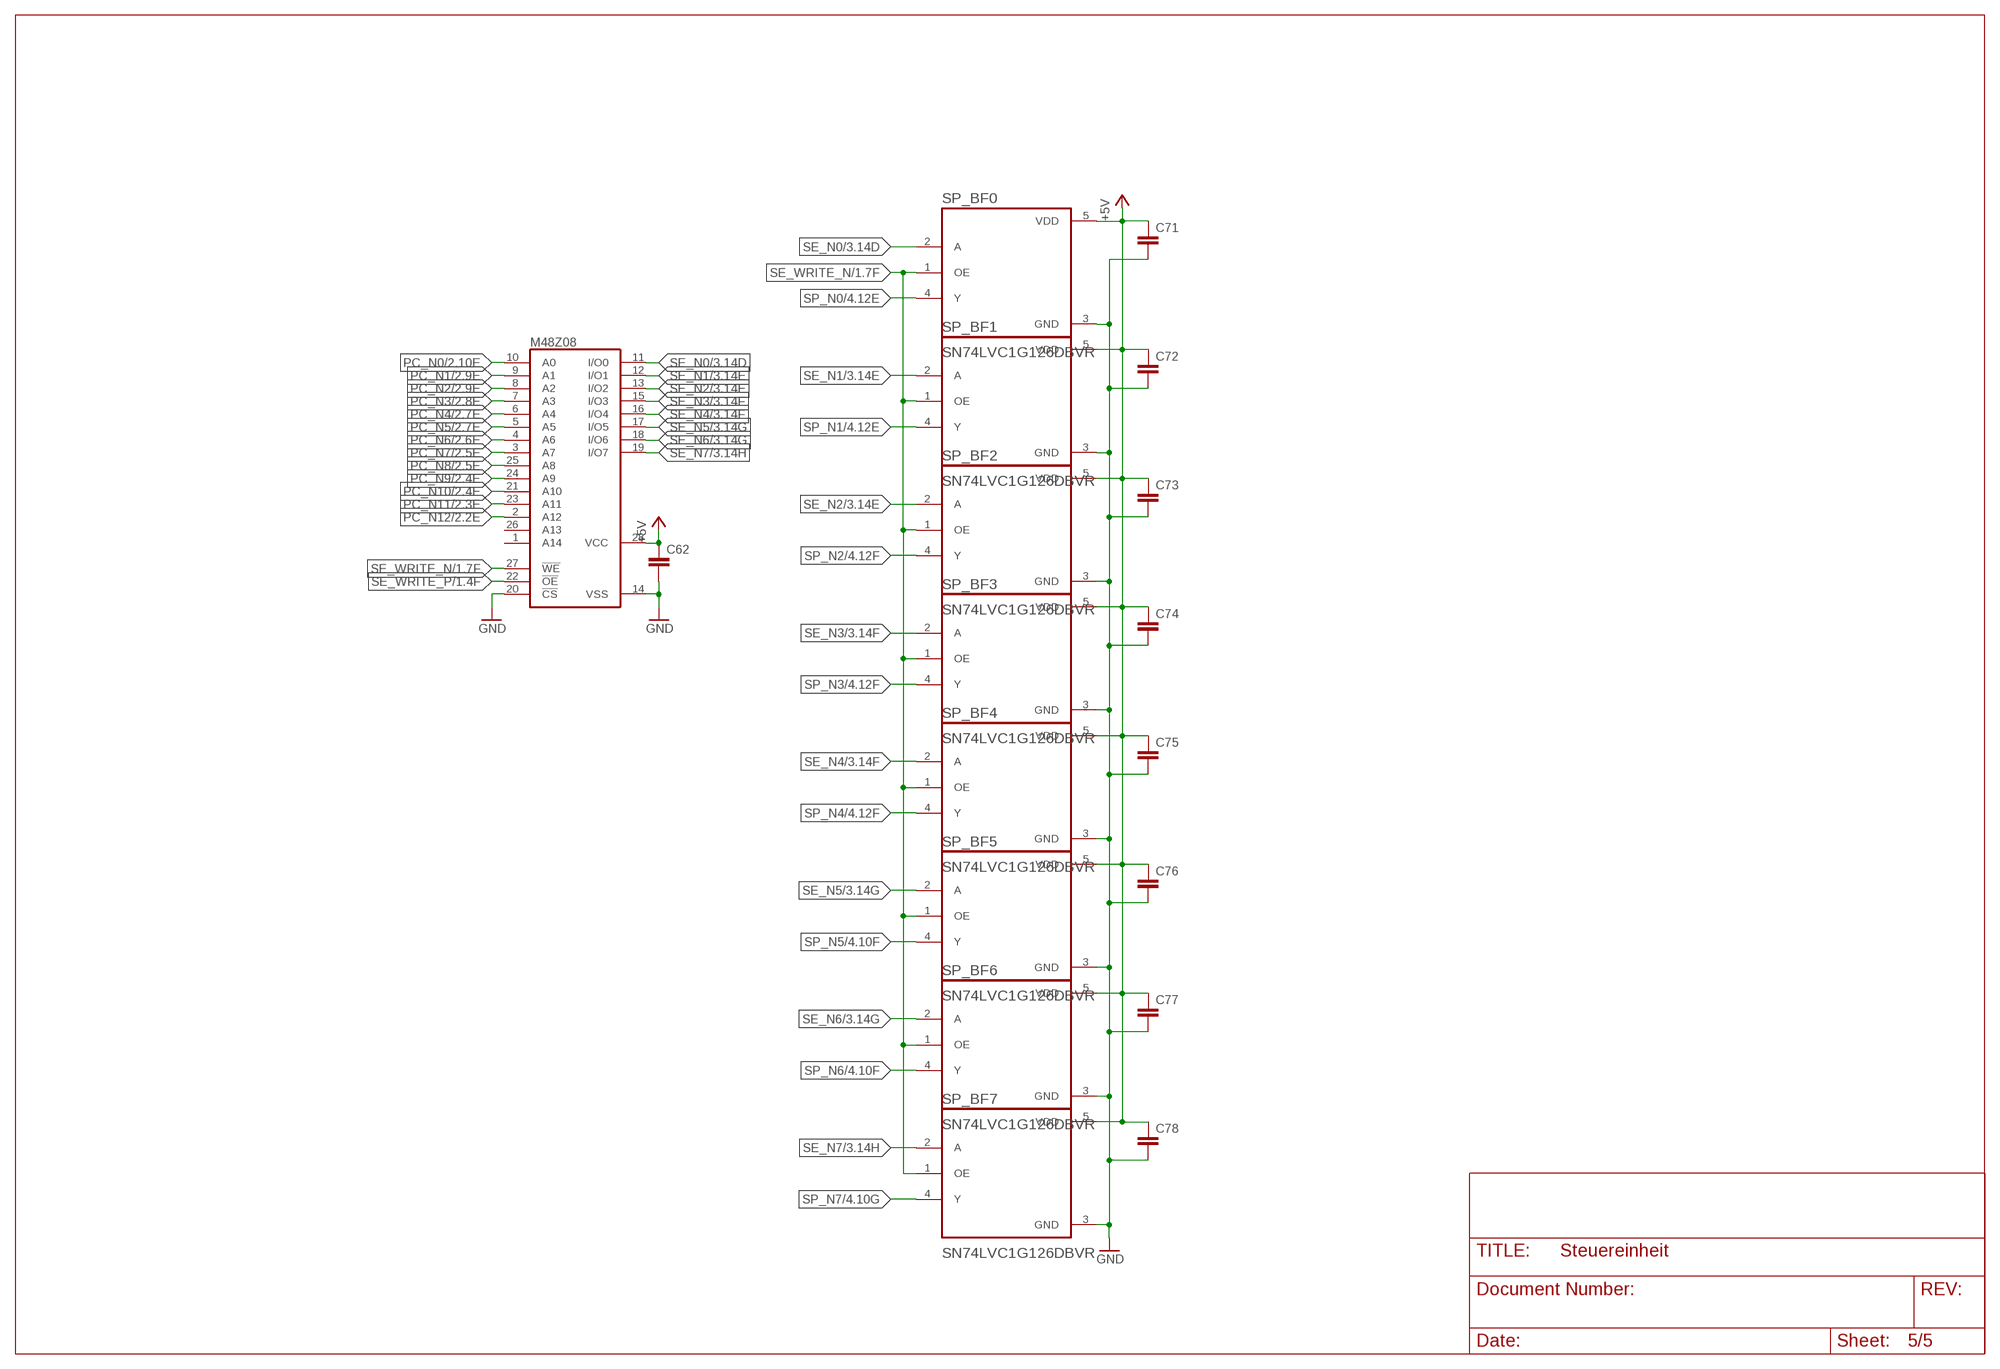
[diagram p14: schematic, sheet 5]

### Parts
C62  C-EUC0805  [C0805]
C71  C-EUC0805  [C0805]
C72  C-EUC0805  [C0805]
C73  C-EUC0805  [C0805]
C74  C-EUC0805  [C0805]
C75  C-EUC0805  [C0805]
C76  C-EUC0805  [C0805]
C77  C-EUC0805  [C0805]
C78  C-EUC0805  [C0805]
M48Z08  62832P1  [DIL28-6]
SP_BF0  SN74LVC1G126DBVR  [SOT95P280X145-5N]
SP_BF1  SN74LVC1G126DBVR  [SOT95P280X145-5N]
SP_BF2  SN74LVC1G126DBVR  [SOT95P280X145-5N]
SP_BF3  SN74LVC1G126DBVR  [SOT95P280X145-5N]
SP_BF4  SN74LVC1G126DBVR  [SOT95P280X145-5N]
SP_BF5  SN74LVC1G126DBVR  [SOT95P280X145-5N]
SP_BF6  SN74LVC1G126DBVR  [SOT95P280X145-5N]
SP_BF7  SN74LVC1G126DBVR  [SOT95P280X145-5N]

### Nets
+5V: C62.1 C71.1 C72.1 C73.1 C74.1 C75.1 C76.1 C77.1 C78.1 M48Z08.28(VCC) SP_BF0.5(VDD) SP_BF1.5(VDD) SP_BF2.5(VDD) SP_BF3.5(VDD) SP_BF4.5(VDD) SP_BF5.5(VDD) SP_BF6.5(VDD) SP_BF7.5(VDD) ; also sheet 1,2,3,4
GND: C62.2 C71.2 C72.2 C73.2 C74.2 C75.2 C76.2 C77.2 C78.2 M48Z08.14(VSS) M48Z08.20(!CS) SP_BF0.3(GND) SP_BF1.3(GND) SP_BF2.3(GND) SP_BF3.3(GND) SP_BF4.3(GND) SP_BF5.3(GND) SP_BF6.3(GND) SP_BF7.3(GND) ; also sheet 1,2,3,4
PC_N0: M48Z08.10(A0) ; also sheet 2
PC_N1: M48Z08.9(A1) ; also sheet 2
PC_N2: M48Z08.8(A2) ; also sheet 2
PC_N3: M48Z08.7(A3) ; also sheet 2
PC_N4: M48Z08.6(A4) ; also sheet 2
PC_N5: M48Z08.5(A5) ; also sheet 2
PC_N6: M48Z08.4(A6) ; also sheet 2
PC_N7: M48Z08.3(A7) ; also sheet 2
PC_N8: M48Z08.25(A8) ; also sheet 2
PC_N9: M48Z08.24(A9) ; also sheet 2
PC_N10: M48Z08.21(A10) ; also sheet 2
PC_N11: M48Z08.23(A11) ; also sheet 2
PC_N12: M48Z08.2(A12) ; also sheet 2
SE_N0: M48Z08.11(I/O0) SP_BF0.2(A) ; also sheet 3
SE_N1: M48Z08.12(I/O1) SP_BF1.2(A) ; also sheet 3
SE_N2: M48Z08.13(I/O2) SP_BF2.2(A) ; also sheet 3
SE_N3: M48Z08.15(I/O3) SP_BF3.2(A) ; also sheet 3
SE_N4: M48Z08.16(I/O4) SP_BF4.2(A) ; also sheet 3
SE_N5: M48Z08.17(I/O5) SP_BF5.2(A) ; also sheet 3
SE_N6: M48Z08.18(I/O6) SP_BF6.2(A) ; also sheet 3
SE_N7: M48Z08.19(I/O7) SP_BF7.2(A) ; also sheet 3
SE_WRITE_N: M48Z08.27(!WE) SP_BF0.1(OE) SP_BF1.1(OE) SP_BF2.1(OE) SP_BF3.1(OE) SP_BF4.1(OE) SP_BF5.1(OE) SP_BF6.1(OE) SP_BF7.1(OE) ; also sheet 1,2,3
SE_WRITE_P: M48Z08.22(!OE) ; also sheet 1,2,3
SP_N0: SP_BF0.4(Y) ; also sheet 4
SP_N1: SP_BF1.4(Y) ; also sheet 4
SP_N2: SP_BF2.4(Y) ; also sheet 4
SP_N3: SP_BF3.4(Y) ; also sheet 4
SP_N4: SP_BF4.4(Y) ; also sheet 4
SP_N5: SP_BF5.4(Y) ; also sheet 4
SP_N6: SP_BF6.4(Y) ; also sheet 4
SP_N7: SP_BF7.4(Y) ; also sheet 4
Unconnected: M48Z08.1(A14) M48Z08.26(A13)

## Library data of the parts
+5V CARRY CHECK CLK GND SMF = pinhead:PINHD-1X1: PIN HEADER
BR_AA1-BR_AA4 = 40xx:4082: Dual 4-input AND
BR_AN1-BR_AN6 PC_AN1-PC_AN11 SE_AN1-SE_AN3 = 40xx:4081: Quad 2-input AND
BR_JK1-BR_JK8 PC_JK1-PC_JK7 SE_JK1-SE_JK12 = 40xx:4027: Dual JK FLIP FLOP
BR_NO1-BR_NO4 M_NO1 PC_NO1 PC_NO2 SE_N01 = 40xx:4049: Hex inverting BUFFER
BR_OR1 BR_OR2 BR_OR4 BR_OR5 M_OR1 = 40xx:4071: Quad 2-input OR
C1-C8 C11-C33 C35-C79 C81-C94 MCLKC PLC = rcl:C-EU: CAPACITOR, European symbol; SPICEPREFIX: C
C9 C10 = deto:C
C_H C_P M_CLK SE_CLK SEN0 SEN1-SEN7 = rcl:R-EU_: RESISTOR, European symbol; SPICEPREFIX: R
CLKNO = 40xx:40106: Hex SCHMITT TRIGGER
COM NU/AD READ REGISTER = pinhead:PINHD-1X4: PIN HEADER
FT232 = deto2:FTDI232: FT232R USB zu RS232 Konverter von FTDI www.ftdichip.com
M48Z08 = memoryMoritz:62832P: MEMORY
MCLKR1 MCLKR2 PLR = rcl:L-EU: INDUCTOR, European symbol; SPICEPREFIX: L
MCLKR3 = pot:TRIM_EU-: POTENTIOMETER
PL_XR = 40xx:4070: Quad 2-input XOR
PLD = diode:1N4446: DIODE
R12 = deto:R: Widerstand 400 mil - 0805 - 1206
RE_BF0 RE_BF1-RE_BF3 SE_BF0 SE_BF1-SE_BF7 SP_BF0 SP_BF1-SP_BF7 WR_BF0 WR_BF1-WR_BF3 = SN74LVC1G126DBVR:SN74LVC1G126DBVR: Check availability; AVAILABILITY: In Stock; CHECK_PRICES: https://www.snapeda.com/parts/SN74LVC1G126DBVR/Texas+Instruments/view-part/?ref=eda; DESCRIPTION: Single 1.65-V to 5.5-V buffer with 3-state outputs; MF: Texas Instruments; MP: SN74LVC1G126DBVR; PACKAGE: SOT-23-5 Texas Instruments; PRICE: None; PURCHASE-URL: https://www.snapeda.com/api/url_track_click_mouser/?unipart_id=184454&manufacturer=Texas Instruments&part_name=SN74LVC1G126DBVR&search_term=None; SNAPEDA_LINK: https://www.snapeda.com/parts/SN74LVC1G126DBVR/Texas+Instruments/view-part/?ref=snap
X2 = con-cypressindustries:MINI-USB-SCHIELD-: MINI USB-B Conector Source: www.cypressindustries.com; OC_FARNELL: unknown; OC_NEWARK: unknown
